//**************************************************************************
//
//   NST_UDT.AWL
//
//   PLC user interface assignment (810D/840D/840Di/FM-NC)
//
//   UDT  2 AL/MSG-UDT
//   UDT 10 NCK-UDT
//   UDT 11 BAG-UDT
//   UDT 19 MMC-UDT
//   UDT 21 Channel UDT
//   UDT 31 Axis/Spindle UDT
//   UDT 77 Mcp
//   UDT 1002 new Alarms
//
//**************************************************************************

//********** FM/BM-UDT **********
TYPE UDT 2


  STRUCT
   C1 : STRUCT  //From Channel 1
    FDD_5100xx : ARRAY  [0 .. 15 ] OF //Feed disable A.no.51000-510015
    BOOL ;
    FDD_RID_5101xx : ARRAY  [0 .. 31 ] OF //Feed and read-in disable A.no.510100-510131
    BOOL ;
    RID_5102xx : ARRAY  [0 .. 31 ] OF //Read-in disable A.no.510200-510231
    BOOL ;
    NCSD_5103xx : ARRAY  [0 .. 15 ] OF //NC start disable A.no.510300-510315
    BOOL ;
    FdStop_1_5111xx : ARRAY  [0 .. 15 ] OF //Feed stop GEOaxis 1 A.no.511100-511115
    BOOL ;
    FdStop_2_5112xx : ARRAY  [0 .. 15 ] OF //Feed stop GEOaxis 2 A.no.511200-511215
    BOOL ;
    FdStop_3_5113xx : ARRAY  [0 .. 15 ] OF //Feed stop GEOaxis 3 A.no.511300-511315
    BOOL ;
   END_STRUCT ;
   C2 : STRUCT  //From Channel 2
    FDD_5200xx : ARRAY  [0 .. 15 ] OF //Feed disable A.no.520000-520015
    BOOL ;
    FDD_RID_5201xx : ARRAY  [0 .. 31 ] OF //Feed and read-in disable A.no.520100-520131
    BOOL ;
    RID_5202xx : ARRAY  [0 .. 31 ] OF //Read-in disable A.no.520200-520231
    BOOL ;
    NCSD_5203xx : ARRAY  [0 .. 15 ] OF //NC start disable A.no.520300-520315
    BOOL ;
    FdStop_1_5211xx : ARRAY  [0 .. 15 ] OF //Feed stop GEOaxis 1 A.no.521100-521115
    BOOL ;
    FdStop_2_5212xx : ARRAY  [0 .. 15 ] OF //Feed stop GEOaxis 2 A.no.521200-521215
    BOOL ;
    FdStop_3_5213xx : ARRAY  [0 .. 15 ] OF //Feed stop GEOaxis 3 A.no.521300-521315
    BOOL ;
   END_STRUCT ;
   C3 : STRUCT  //From Channel 3
    FDD_5300xx : ARRAY  [0 .. 15 ] OF //Feed disable A.no.530000-530015
    BOOL ;
    FDD_RID_5301xx : ARRAY  [0 .. 31 ] OF //Feed and read-in disable A.no.530100-530131
    BOOL ;
    RID_5302xx : ARRAY  [0 .. 31 ] OF //Read-in disable A.no.530200-530231
    BOOL ;
    NCSD_5303xx : ARRAY  [0 .. 15 ] OF //NC start disable A.no.530300-530315
    BOOL ;
    FdStop_1_5311xx : ARRAY  [0 .. 15 ] OF //Feed stop GEOaxis 1 A.no.531100-531115
    BOOL ;
    FdStop_2_5312xx : ARRAY  [0 .. 15 ] OF //Feed stop GEOaxis 2 A.no.531200-531215
    BOOL ;
    FdStop_3_5313xx : ARRAY  [0 .. 15 ] OF //Feed stop GEOaxis 3 A.no.531300-531315
    BOOL ;
   END_STRUCT ;
   C4 : STRUCT  //From Channel 4
    FDD_5400xx : ARRAY  [0 .. 15 ] OF //Feed disable A.no.540000-540015
    BOOL ;
    FDD_RID_5401xx : ARRAY  [0 .. 31 ] OF //Feed and read-in disable A.no.540100-540131
    BOOL ;
    RID_5402xx : ARRAY  [0 .. 31 ] OF //Read-in disable A.no.540200-540231
    BOOL ;
    NCSD_5403xx : ARRAY  [0 .. 15 ] OF //NC start disable A.no.540300-540315
    BOOL ;
    FdStop_1_5411xx : ARRAY  [0 .. 15 ] OF //Feed stop GEOaxis 1 A.no.541100-541115
    BOOL ;
    FdStop_2_5412xx : ARRAY  [0 .. 15 ] OF //Feed stop GEOaxis 2 A.no.541200-541215
    BOOL ;
    FdStop_3_5413xx : ARRAY  [0 .. 15 ] OF //Feed stop GEOaxis 3 A.no.541300-541315
    BOOL ;
   END_STRUCT ;
   C5 : STRUCT  //From Channel 5
    FDD_5500xx : ARRAY  [0 .. 15 ] OF //Feed disable A.no.550000-550015
    BOOL ;
    FDD_RID_5501xx : ARRAY  [0 .. 31 ] OF //Feed and read-in disable A.no.550100-550131
    BOOL ;
    RID_5502xx : ARRAY  [0 .. 31 ] OF //Read-in disable A.no.550200-550231
    BOOL ;
    NCSD_5503xx : ARRAY  [0 .. 15 ] OF //NC start disable A.no.550300-550315
    BOOL ;
    FdStop_1_5511xx : ARRAY  [0 .. 15 ] OF //Feed stop GEOaxis 1 A.no.551100-551115
    BOOL ;
    FdStop_2_5512xx : ARRAY  [0 .. 15 ] OF //Feed stop GEOaxis 2 A.no.551200-551215
    BOOL ;
    FdStop_3_5513xx : ARRAY  [0 .. 15 ] OF //Feed stop GEOaxis 3 A.no.551300-551315
    BOOL ;
   END_STRUCT ;
   C6 : STRUCT  //From Channel 6
    FDD_5600xx : ARRAY  [0 .. 15 ] OF //Feed disable A.no.560000-560015
    BOOL ;
    FDD_RID_5601xx : ARRAY  [0 .. 31 ] OF //Feed and read-in disable A.no.560100-560131
    BOOL ;
    RID_5602xx : ARRAY  [0 .. 31 ] OF //Read-in disable A.no.560200-560231
    BOOL ;
    NCSD_5603xx : ARRAY  [0 .. 15 ] OF //NC start disable A.no.560300-560315
    BOOL ;
    FdStop_1_5611xx : ARRAY  [0 .. 15 ] OF //Feed stop GEOaxis 1 A.no.561100-561115
    BOOL ;
    FdStop_2_5612xx : ARRAY  [0 .. 15 ] OF //Feed stop GEOaxis 2 A.no.561200-561215
    BOOL ;
    FdStop_3_5613xx : ARRAY  [0 .. 15 ] OF //Feed stop GEOaxis 3 A.no.561300-561315
    BOOL ;
   END_STRUCT ;
   C7 : STRUCT  //From Channel 7
    FDD_5700xx : ARRAY  [0 .. 15 ] OF //Feed disable A.no.570000-570015
    BOOL ;
    FDD_RID_5701xx : ARRAY  [0 .. 31 ] OF //Feed and read-in disable A.no.570100-570131
    BOOL ;
    RID_5702xx : ARRAY  [0 .. 31 ] OF //Read-in disable A.no.570200-570231
    BOOL ;
    NCSD_5703xx : ARRAY  [0 .. 15 ] OF //NC start disable A.no.570300-570315
    BOOL ;
    FdStop_1_5711xx : ARRAY  [0 .. 15 ] OF //Feed stop GEOaxis 1 A.no.571100-511115
    BOOL ;
    FdStop_2_5712xx : ARRAY  [0 .. 15 ] OF //Feed stop GEOaxis 2 A.no.571200-511215
    BOOL ;
    FdStop_3_5713xx : ARRAY  [0 .. 15 ] OF //Feed stop GEOaxis 3 A.no.571300-511315
    BOOL ;
   END_STRUCT ;
   C8 : STRUCT  //From Channel 8
    FDD_5800xx : ARRAY  [0 .. 15 ] OF //Feed disable A.no.580000-580015
    BOOL ;
    FDD_RID_5801xx : ARRAY  [0 .. 31 ] OF //Feed and read-in disable A.no.580100-510131
    BOOL ;
    RID_5802xx : ARRAY  [0 .. 31 ] OF //Read-in disable A.no.580200-580231
    BOOL ;
    NCSD_5803xx : ARRAY  [0 .. 15 ] OF //NC start disable A.no.580300-580315
    BOOL ;
    FdStop_1_5811xx : ARRAY  [0 .. 15 ] OF //Feed stop GEOaxis 1 A.no.581100-511115
    BOOL ;
    FdStop_2_5812xx : ARRAY  [0 .. 15 ] OF //Feed stop GEOaxis 2 A.no.581200-511215
    BOOL ;
    FdStop_3_5813xx : ARRAY  [0 .. 15 ] OF //Feed stop GEOaxis 3 A.no.581300-511315
    BOOL ;
   END_STRUCT ;

    _1FdStop6001xx : ARRAY  [0 .. 15 ] OF //Feed stop axis/spindle 1
    BOOL ;
    _2FdStop6002xx : ARRAY  [0 .. 15 ] OF //Feed stop axis/spindle 2
    BOOL ;
    _3FdStop6003xx : ARRAY  [0 .. 15 ] OF //Feed stop axis/spindle 3
    BOOL ;
    _4FdStop6004xx : ARRAY  [0 .. 15 ] OF //Feed stop axis/spindle 4
    BOOL ;
    _5FdStop6005xx : ARRAY  [0 .. 15 ] OF //Feed stop axis/spindle 5
    BOOL ;
    _6FdStop6006xx : ARRAY  [0 .. 15 ] OF //Feed stop axis/spindle 6
    BOOL ;
    _7FdStop6007xx : ARRAY  [0 .. 15 ] OF //Feed stop axis/spindle 7
    BOOL ;
    _8FdStop6008xx : ARRAY  [0 .. 15 ] OF //Feed stop axis/spindle 8
    BOOL ;
    _9FdStop6009xx : ARRAY  [0 .. 15 ] OF //Feed stop axis/spindle 9
    BOOL ;
   _10FdStop6010xx : ARRAY  [0 .. 15 ] OF //Feed stop axis/spindle 10
    BOOL ;
   _11FdStop6011xx : ARRAY  [0 .. 15 ] OF //Feed stop axis/spindle 11
    BOOL ;
   _12FdStop6012xx : ARRAY  [0 .. 15 ] OF //Feed stop axis/spindle 12
    BOOL ;
   _13FdStop6013xx : ARRAY  [0 .. 15 ] OF //Feed stop axis/spindle 13
    BOOL ;
   _14FdStop6014xx : ARRAY  [0 .. 15 ] OF //Feed stop axis/spindle 14
    BOOL ;
   _15FdStop6015xx : ARRAY  [0 .. 15 ] OF //Feed stop axis/spindle 15
    BOOL ;
   _16FdStop6016xx : ARRAY  [0 .. 15 ] OF //Feed stop axis/spindle 16
    BOOL ;
   _17FdStop6017xx : ARRAY  [0 .. 15 ] OF //Feed stop axis/spindle 17
    BOOL ;
   _18FdStop6018xx : ARRAY  [0 .. 15 ] OF //Feed stop axis/spindle 18
    BOOL ;

   A7000xx : ARRAY  [0 .. 63 ] OF //Alarm 700000-700063 (user area 0)
   BOOL ;
   A7001xx : ARRAY  [0 .. 63 ] OF //Alarm 700100-700163 (user area 1)
   BOOL ;
   A7002xx : ARRAY  [0 .. 63 ] OF //Alarm 700200-700263 (user area 2)
   BOOL ;
   A7003xx : ARRAY  [0 .. 63 ] OF //Alarm 700300-700363 (user area 3)
   BOOL ;
   A7004xx : ARRAY  [0 .. 63 ] OF //Alarm 700400-700463 (user area 4)
   BOOL ;
   A7005xx : ARRAY  [0 .. 63 ] OF //Alarm 700500-700563 (user area 5
   BOOL ;
   A7006xx : ARRAY  [0 .. 63 ] OF //Alarm 700600-700663 (user area 6)
   BOOL ;
   A7007xx : ARRAY  [0 .. 63 ] OF //Alarm 700700-700763 (user area 7)
   BOOL ;
   A7008xx : ARRAY  [0 .. 63 ] OF //Alarm 700800-700863 (user area 8)
   BOOL ;
   A7009xx : ARRAY  [0 .. 63 ] OF //Alarm 700900-700963 (user area 9)
   BOOL ;
  END_STRUCT ;




END_TYPE


//********** NCK-UDT **********
TYPE UDT 10

    STRUCT
   A_Disabl_Inp1 : BOOL ;   //Disable digi. NCK input 1
   A_Disabl_Inp2 : BOOL ;   //Disable digi. NCK input 2
   A_Disabl_Inp3 : BOOL ;   //Disable digi. NCK input 3
   A_Disabl_Inp4 : BOOL ;   //Disable digi. NCK input 4
   A_Disabl_Inp5 : BOOL ;   //Disable digi. NCK input 5
   A_Disabl_Inp6 : BOOL ;   //Disable digi. NCK input 6
   A_Disabl_Inp7 : BOOL ;   //Disable digi. NCK input 7
   A_Disabl_Inp8 : BOOL ;   //Disable digi. NCK input 8
   A_Set_Inp1 : BOOL ;  //Set digi. NCK input 1
   A_Set_Inp2 : BOOL ;  //Set digi. NCK input 2
   A_Set_Inp3 : BOOL ;  //Set digi. NCK input 3
   A_Set_Inp4 : BOOL ;  //Set digi. NCK input 4
   A_Set_Inp5 : BOOL ;  //Set digi. NCK input 5
   A_Set_Inp6 : BOOL ;  //Set digi. NCK input 6
   A_Set_Inp7 : BOOL ;  //Set digi. NCK input 7
   A_Set_Inp8 : BOOL ;  //Set digi. NCK input 8
   f0_f15 : ARRAY  [0 .. 15 ] OF BOOL ; //Reserved
   A_Disabl_Out1 : BOOL ;   //Disable digi. NCK output 1
   A_Disabl_Out2 : BOOL ;   //Disable digi. NCK output 2
   A_Disabl_Out3 : BOOL ;   //Disable digi. NCK output 3
   A_Disabl_Out4 : BOOL ;   //Disable digi. NCK output 4
   A_Disabl_Out5 : BOOL ;   //Disable digi. NCK output 5
   A_Disabl_Out6 : BOOL ;   //Disable digi. NCK output 6
   A_Disabl_Out7 : BOOL ;   //Disable digi. NCK output 7
   A_Disabl_Out8 : BOOL ;   //Disable digi. NCK output 8
   A_OvMask_Out1 : BOOL ;   //Overwrite mask of digi. output 1
   A_OvMask_Out2 : BOOL ;   //Overwrite mask of digi. output 2
   A_OvMask_Out3 : BOOL ;   //Overwrite mask of digi. output 3
   A_OvMask_Out4 : BOOL ;   //Overwrite mask of digi. output 4
   A_OvMask_Out5 : BOOL ;   //Overwrite mask of digi. output 5
   A_OvMask_Out6 : BOOL ;   //Overwrite mask of digi. output 6
   A_OvMask_Out7 : BOOL ;   //Overwrite mask of digi. output 7
   A_OvMask_Out8 : BOOL ;   //Overwrite mask of digi. output 8
   A_Set_Out1 : BOOL ;  //Set digi. NCK output 1
   A_Set_Out2 : BOOL ;  //Set digi. NCK output 2
   A_Set_Out3 : BOOL ;  //Set digi. NCK output 3
   A_Set_Out4 : BOOL ;  //Set digi. NCK output 4
   A_Set_Out5 : BOOL ;  //Set digi. NCK output 5
   A_Set_Out6 : BOOL ;  //Set digi. NCK output 6
   A_Set_Out7 : BOOL ;  //Set digi. NCK output 7
   A_Set_Out8 : BOOL ;  //Set digi. NCK output 8
   A_InMask_Out1 : BOOL ;   //Input mask of digi. output 1
   A_InMask_Out2 : BOOL ;   //Input mask of digi. output 2
   A_InMask_Out3 : BOOL ;   //Input mask of digi. output 3
   A_InMask_Out4 : BOOL ;   //Input mask of digi. output 4
   A_InMask_Out5 : BOOL ;   //Input mask of digi. output 5
   A_InMask_Out6 : BOOL ;   //Input mask of digi. output 6
   A_InMask_Out7 : BOOL ;   //Input mask of digi. output 7
   A_InMask_Out8 : BOOL ;   //Input mask of digi. output 8
   MCP1AxisTbl : ARRAY  [1 .. 22 ] OF BYTE := B#16#1,B#16#2,B#16#3,B#16#4,B#16#5,B#16#6,B#16#7,
     B#16#8,B#16#9,B#16#0A,B#16#0B,B#16#0C ;    //Axis No. Table MCP1
   MCP1MaxAxis : Word ; //max. of Axisno, must be smaller or equal gp_par.MaxAxis
   MCP2AxisTbl : ARRAY  [1 .. 22 ] OF BYTE := B#16#1,B#16#2,B#16#3,B#16#4,B#16#5,B#16#6,B#16#7,
     B#16#8,B#16#9,B#16#0A,B#16#0B,B#16#0C ;    //Axis No. Table MCP2
   MCP2MaxAxis : Word ; //max. of Axisno, must be smaller or equal gp_par.MaxAxis
   f56_0 : BOOL ;
   A_EMERGENCY : BOOL ; //Emergency stop
   A_EMERGENCY_Ackn : BOOL ;    //Acknowledge emergency stop
   f56_3 : BOOL ;
   A_Keyswitch0 : BOOL ;    //Keyswitch position 0
   A_Keyswitch1 : BOOL ;    //Keyswitch position 1
   A_Keyswitch2 : BOOL ;    //Keyswitch position 2
   A_Keyswitch3 : BOOL ;    //Keyswitch position 3
   A_IncInModeGroup: BOOL ; //INC inputs in mode group area active
   f57_1 : BOOL ;
   f57_2 : BOOL ;
   A_PCshutdown : BOOL ;    //PC shutdown 840Di
   f57_4 : BOOL ;
   f57_5 : BOOL ;
   f57_6 : BOOL ;
   f57_7 : BOOL ;
   A_CollCheckOff: BOOL ; //Collisions Check Off
   f58_1 : BOOL ;
   f58_2 : BOOL ;
   f58_3 : BOOL ;
   f58_4 : BOOL ;
   f58_5 : BOOL ;
   f58_6 : BOOL ;
   f58_7 : BOOL ;
   f59 : BYTE ;
   E_ActVal_In1 : BOOL ;    //Actual value of digi. NCK input 1
   E_ActVal_In2 : BOOL ;    //Actual value of digi. NCK input 2
   E_ActVal_In3 : BOOL ;    //Actual value of digi. NCK input 3
   E_ActVal_In4 : BOOL ;    //Actual value of digi. NCK input 4
   f60_4 : BOOL ;
   f60_5 : BOOL ;
   f60_6 : BOOL ;
   f60_7 : BOOL ;
   f61_f62 : ARRAY  [61 .. 61 ] OF BYTE ;
   E_Setpoint_Out1 : BOOL ; //Setpoint of digi. NCK output 1
   E_Setpoint_Out2 : BOOL ; //Setpoint of digi. NCK output 2
   E_Setpoint_Out3 : BOOL ; //Setpoint of digi. NCK output 3
   E_Setpoint_Out4 : BOOL ; //Setpoint of digi. NCK output 4
   E_Setpoint_Out5 : BOOL ; //Setpoint of digi. NCK output 5
   E_Setpoint_Out6 : BOOL ; //Setpoint of digi. NCK output 6
   E_Setpoint_Out7 : BOOL ; //Setpoint of digi. NCK output 7
   E_Setpoint_Out8 : BOOL ; //Setpoint of digi. NCK output 8
   f65_f67 : ARRAY  [65 .. 66 ] OF BYTE ;
   E_HW1_moved : BYTE ; //Handwheel 1 moved
   E_HW2_moved : BYTE ; //Handwheel 2 moved
   E_HW3_moved : BYTE ; //Handwheel 3 moved
   E_CounterInchMetr : BYTE ;   //Modification counter inch/metric system of units

   E_MCP1AxisValid :Bool; //from HT6
   E_MCP1WCS :Bool; //from HT6
   f72_2: Bool;
   f72_3: Bool;
   f72_4: Bool;
   f72_5: Bool;
   f72_6: Bool;
   E_MCP1AxKeyDisp: Bool; //Mcp1 Axis Key Displayed
   E_MCP2AxisValid :Bool; //from HT6
   E_MCP2WCS :Bool; //from HT6
   f73_2: Bool;
   f73_3: Bool;
   f73_4: Bool;
   f73_5: Bool;
   f73_6: Bool;
   E_MCP2AxKeyDisp: Bool; //Mcp2 Axis Key Displayed
   MCP1AxisFromHMI : ARRAY [1..6] Of BYTE; //Axistable from HT6
   MCP2AxisFromHMI : ARRAY [1..6] Of BYTE; //Axistable from HT6
   res86 : Word;
   res88 : Byte;
   res89 : Byte;
   epsToPlc: Byte;
   epsFromPlc: Byte;
   MpiDpOk: BOOL;               //Slaves on MPI/DP Ok
   DpOk: BOOL;                  //Slaves on DP Ok
   PnOk : BOOL;                 //Slaves on PN Ok
   f92_3 : BOOL ;
   Disabl_AlarmMpiDp : BOOL;    //Disable Alarmmessage "MPI/DP bus error" (400551)
   Disabl_AlarmDp    : BOOL;    //Disable Alarmmessage "DP bus error" (400552)
   Disabl_AlarmPn    : BOOL;    //Disable Alarmmessage "PN bus error" (400553)
   f92_7 : BOOL ;
   E_CA_AutoMach  : BOOL;     // Disable collision avoidance : AUTO Machine
   E_CA_AutoTools : BOOL;     // Disable collision avoidance : AUTO Tools
   E_CA_AutoWorkh : BOOL;     // Disable collision avoidance : AUTO Workholder
   E_CA_AutoWorkp : BOOL;     // Disable collision avoidance : AUTO Workpieces
   E_CA_JogMach   : BOOL;     // Disable collision avoidance : JOG Machine
   E_CA_JogTools  : BOOL;     // Disable collision avoidance : JOG Tools
   E_CA_JogWorkh  : BOOL;     // Disable collision avoidance : JOG Workholder
   E_CA_JogWorkp  : BOOL;     // Disable collision avoidance : JOG Workpieces
   f94: BYTE ;
   f95: BYTE ;
   E_LanguageID : BYTE ;   // LanguageID on HMI
   E_Chan_HW1_A : BOOL ;    //Channel number for handwheel1 A
   E_Chan_HW1_B : BOOL ;    //Channel number for handwheel1 B
   E_Chan_HW1_C : BOOL ;    //Channel number for handwheel1 C
   E_Chan_HW1_D : BOOL ;    //Channel number for handwheel1 D
   f97_4 : BOOL ;
   f97_5 : BOOL ;
   f97_6 : BOOL ;
   f97_7 : BOOL ;
   E_Chan_HW2_A : BOOL ;    //Channel number for handwheel2 A
   E_Chan_HW2_B : BOOL ;    //Channel number for handwheel2 B
   E_Chan_HW2_C : BOOL ;    //Channel number for handwheel2 C
   E_Chan_HW2_D : BOOL ;    //Channel number for handwheel2 D
   f98_4 : BOOL ;
   f98_5 : BOOL ;
   f98_6 : BOOL ;
   f98_7 : BOOL ;
   E_Chan_HW3_A : BOOL ;    //Channel number for handwheel3 A
   E_Chan_HW3_B : BOOL ;    //Channel number for handwheel3 B
   E_Chan_HW3_C : BOOL ;    //Channel number for handwheel3 C
   E_Chan_HW3_D : BOOL ;    //Channel number for handwheel3 D
   f99_4 : BOOL ;
   f99_5 : BOOL ;
   f99_6 : BOOL ;
   f99_7 : BOOL ;
   E_Ax_A_HW1 : BOOL ;  //Axis number for handwheel1 A
   E_Ax_B_HW1 : BOOL ;  //Axis number for handwheel1 B
   E_Ax_C_HW1 : BOOL ;  //Axis number for handwheel1 C
   E_Ax_D_HW1 : BOOL ;  //Axis number for handwheel1 D
   E_Ax_E_HW1 : BOOL ;  //Axis number for handwheel1 E
   E_CHW_sel1 : BOOL ;  //Contour handwheel selected
   E_HW_sel1 : BOOL ;   //Handwheel selected
   E_Mach_Ax1 : BOOL ;  //Machine axis
   E_Ax_A_HW2 : BOOL ;  //Axis number for handwheel2 A
   E_Ax_B_HW2 : BOOL ;  //Axis number for handwheel2 B
   E_Ax_C_HW2 : BOOL ;  //Axis number for handwheel2 C
   E_Ax_D_HW2 : BOOL ;  //Axis number for handwheel2 D
   E_Ax_E_HW2 : BOOL ;  //Axis number for handwheel2 E
   E_CHW_sel2 : BOOL ;  //Contour handwheel selected
   E_HW_sel2 : BOOL ;   //Handwheel selected
   E_Mach_Ax2 : BOOL ;  //Machine axis
   E_Ax_A_HW3 : BOOL ;  //Axis number for handwheel3 A
   E_Ax_B_HW3 : BOOL ;  //Axis number for handwheel3 B
   E_Ax_C_HW3 : BOOL ;  //Axis number for handwheel3 C
   E_Ax_D_HW3 : BOOL ;  //Axis number for handwheel3 D
   E_Ax_E_HW3 : BOOL ;  //Axis number for handwheel3 E
   E_CHW_sel3 : BOOL ;  //Contour handwheel selected
   E_HW_sel3 : BOOL ;   //Handwheel selected
   E_Mach_Ax3 : BOOL ;  //Machine axis
   E_RemDiag : BOOL ;   //Remote Diagnostic
   f103_1 : BOOL ;
   f103_2 : BOOL ;
   f103_3 : BOOL ;
   f103_4 : BOOL ;
   E_ATready : BOOL ;   //AT-box ready
   E_MMCTemp : BOOL ;   //MMC temperature limit
   E_MMCBatt : BOOL ;   //MMC 101/102 battery alarm
   E_MCP1ready : BOOL ; //MCP1 ready;
   E_MCP2ready : BOOL ; //MCP2 ready;
   E_BHGready : BOOL ;  //BHG ready;
   f104_3 : BOOL ;
   f104_4 : BOOL ;
   f104_5 : BOOL ;
   E_FirstOB1 : BOOL ;  //This bit is on for the first OB1 cycle
   E_NCKready : BOOL ;  //NCK CPU ready
   E_CancelToolCmd : BOOL; //Terminate canceled tool command
   f105_1   : BOOL;
   f105_2   : BOOL;
   f105_3   : BOOL;
   f105_4   : BOOL;
   f105_5   : BOOL;
   f105_6   : BOOL;
   f105_7   : BOOL;
   E_CollCheckOff : BOOL ;  //CollisionsCheck Off
   E_EMSTOP : BOOL ;    //EMERGENCY STOP active
   f106_2 : BOOL ;
   f106_3 : BOOL ;
   f106_4 : BOOL ;
   f106_5 : BOOL ;
   f106_6 : BOOL ;
   f106_7 : BOOL ;
   E_InspProbe1 : BOOL ;    //Inspection probe 1 actuated
   E_InspProbe2 : BOOL ;    //Inspection probe 2 actuated
   f107_2 : BOOL ;
   f107_3 : BOOL ;
   f107_4 : BOOL ;
   f107_5 : BOOL ;
   E_NCU_LinkActive : BOOL ;    //NCU link active
   E_SystemInchDim : BOOL ; //System inch dimension
   f108_0 : BOOL ;
   E_MMC2Ready : BOOL ;     //MMC2-CPU ready
   E_MMCMPIready : BOOL ;   //MMC1-CPU on MPI ready
   E_MMCBTSSready : BOOL ;  //MMC1-CPU on BTSS ready
   f108_4 : BOOL ;
   E_DrivesInCylOp : BOOL ; //Drives in cylindric operation
   E_611Dready : BOOL ; //611D ready
   E_NCready : BOOL ;
   E_NCKalarm : BOOL ;  //NCK alarm present
   f109_1 : BOOL ;
   f109_2 : BOOL ;
   f109_3 : BOOL ;
   A_PC_OSfault : BOOL ;    //PC operating system fault, 840Di
   E_HTempAlarm : BOOL ;    //Heat sink temperature alarm NCU 573
   E_ATempAlarm : BOOL ;    //Air temperature alarm
   E_BattAlarm : BOOL ; //NCK battery alarm
   E_SWCamMinus : ARRAY  [0 .. 31 ] OF BOOL ;   //Software cams minus [0..31]
   E_SWCamPlus : ARRAY  [0 .. 31 ] OF BOOL ;    //Software cams plus [0..31]
   f118_f121 : ARRAY  [0 .. 3 ] OF BYTE ;
   A_Disabl_Inp9 : BOOL ;   //Disable digi. NCK input 9
   A_Disabl_Inp10 : BOOL ;  //Disable digi. NCK input 10
   A_Disabl_Inp11 : BOOL ;  //Disable digi. NCK input 11
   A_Disabl_Inp12 : BOOL ;  //Disable digi. NCK input 12
   A_Disabl_Inp13 : BOOL ;  //Disable digi. NCK input 13
   A_Disabl_Inp14 : BOOL ;  //Disable digi. NCK input 14
   A_Disabl_Inp15 : BOOL ;  //Disable digi. NCK input 15
   A_Disabl_Inp16 : BOOL ;  //Disable digi. NCK input 16
   A_Set_Inp9 : BOOL ;  //Set digi. NCK input 9
   A_Set_Inp10 : BOOL ; //Set digi. NCK input 10
   A_Set_Inp11 : BOOL ; //Set digi. NCK input 11
   A_Set_Inp12 : BOOL ; //Set digi. NCK input 12
   A_Set_Inp13 : BOOL ; //Set digi. NCK input 13
   A_Set_Inp14 : BOOL ; //Set digi. NCK input 14
   A_Set_Inp15 : BOOL ; //Set digi. NCK input 15
   A_Set_Inp16 : BOOL ; //Set digi. NCK input 16
   A_Disabl_Inp17 : BOOL ;  //Disable digi. NCK input 17
   A_Disabl_Inp18 : BOOL ;  //Disable digi. NCK input 18
   A_Disabl_Inp19 : BOOL ;  //Disable digi. NCK input 19
   A_Disabl_Inp20 : BOOL ;  //Disable digi. NCK input 20
   A_Disabl_Inp21 : BOOL ;  //Disable digi. NCK input 21
   A_Disabl_Inp22 : BOOL ;  //Disable digi. NCK input 22
   A_Disabl_Inp23 : BOOL ;  //Disable digi. NCK input 23
   A_Disabl_Inp24 : BOOL ;  //Disable digi. NCK input 24
   A_Set_Inp17 : BOOL ; //Set digi. NCK input 17
   A_Set_Inp18 : BOOL ; //Set digi. NCK input 18
   A_Set_Inp19 : BOOL ; //Set digi. NCK input 19
   A_Set_Inp20 : BOOL ; //Set digi. NCK input 20
   A_Set_Inp21 : BOOL ; //Set digi. NCK input 21
   A_Set_Inp22 : BOOL ; //Set digi. NCK input 22
   A_Set_Inp23 : BOOL ; //Set digi. NCK input 23
   A_Set_Inp24 : BOOL ; //Set digi. NCK input 24
   A_Disabl_Inp25 : BOOL ;  //Disable digi. NCK input 25
   A_Disabl_Inp26 : BOOL ;  //Disable digi. NCK input 26
   A_Disabl_Inp27 : BOOL ;  //Disable digi. NCK input 27
   A_Disabl_Inp28 : BOOL ;  //Disable digi. NCK input 28
   A_Disabl_Inp29 : BOOL ;  //Disable digi. NCK input 29
   A_Disabl_Inp30 : BOOL ;  //Disable digi. NCK input 30
   A_Disabl_Inp31 : BOOL ;  //Disable digi. NCK input 31
   A_Disabl_Inp32 : BOOL ;  //Disable digi. NCK input 32
   A_Set_Inp25 : BOOL ; //Set digi. NCK input 25
   A_Set_Inp26 : BOOL ; //Set digi. NCK input 26
   A_Set_Inp27 : BOOL ; //Set digi. NCK input 27
   A_Set_Inp28 : BOOL ; //Set digi. NCK input 28
   A_Set_Inp29 : BOOL ; //Set digi. NCK input 29
   A_Set_Inp30 : BOOL ; //Set digi. NCK input 30
   A_Set_Inp31 : BOOL ; //Set digi. NCK input 31
   A_Set_Inp32 : BOOL ; //Set digi. NCK input 32
   A_Disabl_Inp33 : BOOL ;  //Disable digi. NCK input 33
   A_Disabl_Inp34 : BOOL ;  //Disable digi. NCK input 34
   A_Disabl_Inp35 : BOOL ;  //Disable digi. NCK input 35
   A_Disabl_Inp36 : BOOL ;  //Disable digi. NCK input 36
   A_Disabl_Inp37 : BOOL ;  //Disable digi. NCK input 37
   A_Disabl_Inp38 : BOOL ;  //Disable digi. NCK input 38
   A_Disabl_Inp39 : BOOL ;  //Disable digi. NCK input 39
   A_Disabl_Inp40 : BOOL ;  //Disable digi. NCK input 40
   A_Set_Inp33 : BOOL ; //Set digi. NCK input 33
   A_Set_Inp34 : BOOL ; //Set digi. NCK input 34
   A_Set_Inp35 : BOOL ; //Set digi. NCK input 35
   A_Set_Inp36 : BOOL ; //Set digi. NCK input 36
   A_Set_Inp37 : BOOL ; //Set digi. NCK input 37
   A_Set_Inp38 : BOOL ; //Set digi. NCK input 38
   A_Set_Inp39 : BOOL ; //Set digi. NCK input 39
   A_Set_Inp40 : BOOL ; //Set digi. NCK input 40
   A_Disabl_Out9 : BOOL ;   //Disable digi. NCK output 9
   A_Disabl_Out10 : BOOL ;  //Disable digi. NCK output 10
   A_Disabl_Out11 : BOOL ;  //Disable digi. NCK output 11
   A_Disabl_Out12 : BOOL ;  //Disable digi. NCK output 12
   A_Disabl_Out13 : BOOL ;  //Disable digi. NCK output 13
   A_Disabl_Out14 : BOOL ;  //Disable digi. NCK output 14
   A_Disabl_Out15 : BOOL ;  //Disable digi. NCK output 15
   A_Disabl_Out16 : BOOL ;  //Disable digi. NCK output 16
   A_OvMask_Out9 : BOOL ;   //Overwrite mask of digi. output 9
   A_OvMask_Out10 : BOOL ;  //Overwrite mask of digi. output 10
   A_OvMask_Out11 : BOOL ;  //Overwrite mask of digi. output 11
   A_OvMask_Out12 : BOOL ;  //Overwrite mask of digi. output 12
   A_OvMask_Out13 : BOOL ;  //Overwrite mask of digi. output 13
   A_OvMask_Out14 : BOOL ;  //Overwrite mask of digi. output 14
   A_OvMask_Out15 : BOOL ;  //Overwrite mask of digi. output 15
   A_OvMask_Out16 : BOOL ;  //Overwrite mask of digi. output 16
   A_Setval_Out9 : BOOL ;   //Set value digi. NCK output 9
   A_Setval_Out10 : BOOL ;  //Set value digi. NCK output 10
   A_Setval_Out11 : BOOL ;  //Set value digi. NCK output 11
   A_Setval_Out12 : BOOL ;  //Set value digi. NCK output 12
   A_Setval_Out13 : BOOL ;  //Set value digi. NCK output 13
   A_Setval_Out14 : BOOL ;  //Set value digi. NCK output 14
   A_Setval_Out15 : BOOL ;  //Set value digi. NCK output 15
   A_Setval_Out16 : BOOL ;  //Set value digi. NCK output 16
   A_InMask_Out9 : BOOL ;   //Input mask of digi. output 9
   A_InMask_Out10 : BOOL ;  //Input mask of digi. output 10
   A_InMask_Out11 : BOOL ;  //Input mask of digi. output 11
   A_InMask_Out12 : BOOL ;  //Input mask of digi. output 12
   A_InMask_Out13 : BOOL ;  //Input mask of digi. output 13
   A_InMask_Out14 : BOOL ;  //Input mask of digi. output 14
   A_InMask_Out15 : BOOL ;  //Input mask of digi. output 15
   A_InMask_Out16 : BOOL ;  //Input mask of digi. output 16
   A_Disabl_Out17 : BOOL ;  //Disable digi. NCK output 17
   A_Disabl_Out18 : BOOL ;  //Disable digi. NCK output 18
   A_Disabl_Out19 : BOOL ;  //Disable digi. NCK output 19
   A_Disabl_Out20 : BOOL ;  //Disable digi. NCK output 20
   A_Disabl_Out21 : BOOL ;  //Disable digi. NCK output 21
   A_Disabl_Out22 : BOOL ;  //Disable digi. NCK output 22
   A_Disabl_Out23 : BOOL ;  //Disable digi. NCK output 23
   A_Disabl_Out24 : BOOL ;  //Disable digi. NCK output 24
   A_OvMask_Out17 : BOOL ;  //Overwrite mask of digi. output 17
   A_OvMask_Out18 : BOOL ;  //Overwrite mask of digi. output 18
   A_OvMask_Out19 : BOOL ;  //Overwrite mask of digi. output 19
   A_OvMask_Out20 : BOOL ;  //Overwrite mask of digi. output 20
   A_OvMask_Out21 : BOOL ;  //Overwrite mask of digi. output 21
   A_OvMask_Out22 : BOOL ;  //Overwrite mask of digi. output 22
   A_OvMask_Out23 : BOOL ;  //Overwrite mask of digi. output 23
   A_OvMask_Out24 : BOOL ;  //Overwrite mask of digi. output 24
   A_Setval_Out17 : BOOL ;  //Set value digi. NCK output 17
   A_Setval_Out18 : BOOL ;  //Set value digi. NCK output 18
   A_Setval_Out19 : BOOL ;  //Set value digi. NCK output 19
   A_Setval_Out20 : BOOL ;  //Set value digi. NCK output 20
   A_Setval_Out21 : BOOL ;  //Set value digi. NCK output 21
   A_Setval_Out22 : BOOL ;  //Set value digi. NCK output 22
   A_Setval_Out23 : BOOL ;  //Set value digi. NCK output 23
   A_Setval_Out24 : BOOL ;  //Set value digi. NCK output 24
   A_InMask_Out17 : BOOL ;  //Input mask of digi. output 17
   A_InMask_Out18 : BOOL ;  //Input mask of digi. output 18
   A_InMask_Out19 : BOOL ;  //Input mask of digi. output 19
   A_InMask_Out20 : BOOL ;  //Input mask of digi. output 20
   A_InMask_Out21 : BOOL ;  //Input mask of digi. output 21
   A_InMask_Out22 : BOOL ;  //Input mask of digi. output 22
   A_InMask_Out23 : BOOL ;  //Input mask of digi. output 23
   A_InMask_Out24 : BOOL ;  //Input mask of digi. output 24
   A_Disabl_Out25 : BOOL ;  //Disable digi. NCK output 25
   A_Disabl_Out26 : BOOL ;  //Disable digi. NCK output 26
   A_Disabl_Out27 : BOOL ;  //Disable digi. NCK output 27
   A_Disabl_Out28 : BOOL ;  //Disable digi. NCK output 28
   A_Disabl_Out29 : BOOL ;  //Disable digi. NCK output 29
   A_Disabl_Out30 : BOOL ;  //Disable digi. NCK output 30
   A_Disabl_Out31 : BOOL ;  //Disable digi. NCK output 31
   A_Disabl_Out32 : BOOL ;  //Disable digi. NCK output 32
   A_OvMask_Out25 : BOOL ;  //Overwrite mask of digi. output 25
   A_OvMask_Out26 : BOOL ;  //Overwrite mask of digi. output 26
   A_OvMask_Out27 : BOOL ;  //Overwrite mask of digi. output 27
   A_OvMask_Out28 : BOOL ;  //Overwrite mask of digi. output 28
   A_OvMask_Out29 : BOOL ;  //Overwrite mask of digi. output 29
   A_OvMask_Out30 : BOOL ;  //Overwrite mask of digi. output 30
   A_OvMask_Out31 : BOOL ;  //Overwrite mask of digi. output 31
   A_OvMask_Out32 : BOOL ;  //Overwrite mask of digi. output 32
   A_Setval_Out25 : BOOL ;  //Set value digi. NCK output 25
   A_Setval_Out26 : BOOL ;  //Set value digi. NCK output 26
   A_Setval_Out27 : BOOL ;  //Set value digi. NCK output 27
   A_Setval_Out28 : BOOL ;  //Set value digi. NCK output 28
   A_Setval_Out29 : BOOL ;  //Set value digi. NCK output 29
   A_Setval_Out30 : BOOL ;  //Set value digi. NCK output 30
   A_Setval_Out31 : BOOL ;  //Set value digi. NCK output 31
   A_Setval_Out32 : BOOL ;  //Set value digi. NCK output 32
   A_InMask_Out25 : BOOL ;  //Input mask of digi. output 25
   A_InMask_Out26 : BOOL ;  //Input mask of digi. output 26
   A_InMask_Out27 : BOOL ;  //Input mask of digi. output 27
   A_InMask_Out28 : BOOL ;  //Input mask of digi. output 28
   A_InMask_Out29 : BOOL ;  //Input mask of digi. output 29
   A_InMask_Out30 : BOOL ;  //Input mask of digi. output 30
   A_InMask_Out31 : BOOL ;  //Input mask of digi. output 31
   A_InMask_Out32 : BOOL ;  //Input mask of digi. output 32
   A_Disabl_Out33 : BOOL ;  //Disable digi. NCK output 33
   A_Disabl_Out34 : BOOL ;  //Disable digi. NCK output 34
   A_Disabl_Out35 : BOOL ;  //Disable digi. NCK output 35
   A_Disabl_Out36 : BOOL ;  //Disable digi. NCK output 36
   A_Disabl_Out37 : BOOL ;  //Disable digi. NCK output 37
   A_Disabl_Out38 : BOOL ;  //Disable digi. NCK output 38
   A_Disabl_Out39 : BOOL ;  //Disable digi. NCK output 39
   A_Disabl_Out40 : BOOL ;  //Disable digi. NCK output 40
   A_OvMask_Out33 : BOOL ;  //Overwrite mask of digi. output 33
   A_OvMask_Out34 : BOOL ;  //Overwrite mask of digi. output 34
   A_OvMask_Out35 : BOOL ;  //Overwrite mask of digi. output 35
   A_OvMask_Out36 : BOOL ;  //Overwrite mask of digi. output 36
   A_OvMask_Out37 : BOOL ;  //Overwrite mask of digi. output 37
   A_OvMask_Out38 : BOOL ;  //Overwrite mask of digi. output 38
   A_OvMask_Out39 : BOOL ;  //Overwrite mask of digi. output 39
   A_OvMask_Out40 : BOOL ;  //Overwrite mask of digi. output 40
   A_Setval_out33 : BOOL ;  //Set value digi. NCK output 33
   A_Setval_out34 : BOOL ;  //Set value digi. NCK output 34
   A_Setval_out35 : BOOL ;  //Set value digi. NCK output 35
   A_Setval_out36 : BOOL ;  //Set value digi. NCK output 36
   A_Setval_out37 : BOOL ;  //Set value digi. NCK output 37
   A_Setval_out38 : BOOL ;  //Set value digi. NCK output 38
   A_Setval_out39 : BOOL ;  //Set value digi. NCK output 39
   A_Setval_out40 : BOOL ;  //Set value digi. NCK output 40
   A_InMask_Out33 : BOOL ;  //Input mask of digi. output 33
   A_InMask_Out34 : BOOL ;  //Input mask of digi. output 34
   A_InMask_Out35 : BOOL ;  //Input mask of digi. output 35
   A_InMask_Out36 : BOOL ;  //Input mask of digi. output 36
   A_InMask_Out37 : BOOL ;  //Input mask of digi. output 37
   A_InMask_Out38 : BOOL ;  //Input mask of digi. output 38
   A_InMask_Out39 : BOOL ;  //Input mask of digi. output 39
   A_InMask_Out40 : BOOL ;  //Input mask of digi. output 40
   A_Disabl_anaIn1 : BOOL ; //Disable analog NCK input 1
   A_Disabl_anaIn2 : BOOL ; //Disable analog NCK input 2
   A_Disabl_anaIn3 : BOOL ; //Disable analog NCK input 3
   A_Disabl_anaIn4 : BOOL ; //Disable analog NCK input 4
   A_Disabl_anaIn5 : BOOL ; //Disable analog NCK input 5
   A_Disabl_anaIn6 : BOOL ; //Disable analog NCK input 6
   A_Disabl_anaIn7 : BOOL ; //Disable analog NCK input 7
   A_Disabl_anaIn8 : BOOL ; //Disable analog NCK input 8
   A_InMask_anaIn1 : BOOL ; //Input mask of analog NCK input 1
   A_InMask_anaIn2 : BOOL ; //Input mask of analog NCK input 2
   A_InMask_anaIn3 : BOOL ; //Input mask of analog NCK input 3
   A_InMask_anaIn4 : BOOL ; //Input mask of analog NCK input 4
   A_InMask_anaIn5 : BOOL ; //Input mask of analog NCK input 5
   A_InMask_anaIn6 : BOOL ; //Input mask of analog NCK input 6
   A_InMask_anaIn7 : BOOL ; //Input mask of analog NCK input 7
   A_InMask_anaIn8 : BOOL ; //Input mask of analog NCK input 8
   A_Setval_anaIn1 : WORD ; //Set value of analog NCK input 1
   A_Setval_anaIn2 : WORD ; //Set value of analog NCK input 2
   A_Setval_anaIn3 : WORD ; //Set value of analog NCK input 3
   A_Setval_anaIn4 : WORD ; //Set value of analog NCK input 4
   A_Setval_anaIn5 : WORD ; //Set value of analog NCK input 5
   A_Setval_anaIn6 : WORD ; //Set value of analog NCK input 6
   A_Setval_anaIn7 : WORD ; //Set value of analog NCK input 7
   A_Setval_anaIn8 : WORD ; //Set value of analog NCK input 8
   f164_f165 : INT ;
   A_OvMask_anaOut1 : BOOL ;    //Overwrite mask of analog output 1
   A_OvMask_anaOut2 : BOOL ;    //Overwrite mask of analog output 2
   A_OvMask_anaOut3 : BOOL ;    //Overwrite mask of analog output 3
   A_OvMask_anaOut4 : BOOL ;    //Overwrite mask of analog output 4
   A_OvMask_anaOut5 : BOOL ;    //Overwrite mask of analog output 5
   A_OvMask_anaOut6 : BOOL ;    //Overwrite mask of analog output 6
   A_OvMask_anaOut7 : BOOL ;    //Overwrite mask of analog output 7
   A_OvMask_anaOut8 : BOOL ;    //Overwrite mask of analog output 8
   A_InMask_anaOut1 : BOOL ;    //Input mask of analog NCK output 1
   A_InMask_anaOut2 : BOOL ;    //Input mask of analog NCK output 2
   A_InMask_anaOut3 : BOOL ;    //Input mask of analog NCK output 3
   A_InMask_anaOut4 : BOOL ;    //Input mask of analog NCK output 4
   A_InMask_anaOut5 : BOOL ;    //Input mask of analog NCK output 5
   A_InMask_anaOut6 : BOOL ;    //Input mask of analog NCK output 6
   A_InMask_anaOut7 : BOOL ;    //Input mask of analog NCK output 7
   A_InMask_anaOut8 : BOOL ;    //Input mask of analog NCK output 8
   A_Disabl_anaOut1 : BOOL ;    //Disable analog NCK output 1
   A_Disabl_anaOut2 : BOOL ;    //Disable analog NCK output 2
   A_Disabl_anaOut3 : BOOL ;    //Disable analog NCK output 3
   A_Disabl_anaOut4 : BOOL ;    //Disable analog NCK output 4
   A_Disabl_anaOut5 : BOOL ;    //Disable analog NCK output 5
   A_Disabl_anaOut6 : BOOL ;    //Disable analog NCK output 6
   A_Disabl_anaOut7 : BOOL ;    //Disable analog NCK output 7
   A_Disabl_anaOut8 : BOOL ;    //Disable analog NCK output 8
   f169 : BYTE ;
   A_Setval_anaOut1 : WORD ;    //Set value of analog NCK output 1
   A_Setval_anaOut2 : WORD ;    //Set value of analog NCK output 2
   A_Setval_anaOut3 : WORD ;    //Set value of analog NCK output 3
   A_Setval_anaOut4 : WORD ;    //Set value of analog NCK output 4
   A_Setval_anaOut5 : WORD ;    //Set value of analog NCK output 5
   A_Setval_anaOut6 : WORD ;    //Set value of analog NCK output 6
   A_Setval_anaOut7 : WORD ;    //Set value of analog NCK output 7
   A_Setval_anaOut8 : WORD ;    //Set value of analog NCK output 8
   E_ActVal_In9 : BOOL ;    //Actual value of digi. NCK input 9
   E_ActVal_In10 : BOOL ;   //Actual value of digi. NCK input 10
   E_ActVal_In11 : BOOL ;   //Actual value of digi. NCK input 11
   E_ActVal_In12 : BOOL ;   //Actual value of digi. NCK input 12
   E_ActVal_In13 : BOOL ;   //Actual value of digi. NCK input 13
   E_ActVal_In14 : BOOL ;   //Actual value of digi. NCK input 14
   E_ActVal_In15 : BOOL ;   //Actual value of digi. NCK input 15
   E_ActVal_In16 : BOOL ;   //Actual value of digi. NCK input 16
   E_ActVal_In17 : BOOL ;   //Actual value of digi. NCK input 17
   E_ActVal_In18 : BOOL ;   //Actual value of digi. NCK input 18
   E_ActVal_In19 : BOOL ;   //Actual value of digi. NCK input 19
   E_ActVal_In20 : BOOL ;   //Actual value of digi. NCK input 20
   E_ActVal_In21 : BOOL ;   //Actual value of digi. NCK input 21
   E_ActVal_In22 : BOOL ;   //Actual value of digi. NCK input 22
   E_ActVal_In23 : BOOL ;   //Actual value of digi. NCK input 23
   E_ActVal_In24 : BOOL ;   //Actual value of digi. NCK input 24
   E_ActVal_In25 : BOOL ;   //Actual value of digi. NCK input 25
   E_ActVal_In26 : BOOL ;   //Actual value of digi. NCK input 26
   E_ActVal_In27 : BOOL ;   //Actual value of digi. NCK input 27
   E_ActVal_In28 : BOOL ;   //Actual value of digi. NCK input 28
   E_ActVal_In29 : BOOL ;   //Actual value of digi. NCK input 29
   E_ActVal_In30 : BOOL ;   //Actual value of digi. NCK input 30
   E_ActVal_In31 : BOOL ;   //Actual value of digi. NCK input 31
   E_ActVal_In32 : BOOL ;   //Actual value of digi. NCK input 32
   E_ActVal_In33 : BOOL ;   //Actual value of digi. NCK input 33
   E_ActVal_In34 : BOOL ;   //Actual value of digi. NCK input 34
   E_ActVal_In35 : BOOL ;   //Actual value of digi. NCK input 35
   E_ActVal_In36 : BOOL ;   //Actual value of digi. NCK input 36
   E_ActVal_In37 : BOOL ;   //Actual value of digi. NCK input 37
   E_ActVal_In38 : BOOL ;   //Actual value of digi. NCK input 38
   E_ActVal_In39 : BOOL ;   //Actual value of digi. NCK input 39
   E_ActVal_In40 : BOOL ;   //Actual value of digi. NCK input 40
   E_Setpoint_Out9 : BOOL ; //Setpoint of digi. NCK output 9
   E_Setpoint_Out10 : BOOL ;    //Setpoint of digi. NCK output 10
   E_Setpoint_Out11 : BOOL ;    //Setpoint of digi. NCK output 11
   E_Setpoint_Out12 : BOOL ;    //Setpoint of digi. NCK output 12
   E_Setpoint_Out13 : BOOL ;    //Setpoint of digi. NCK output 13
   E_Setpoint_Out14 : BOOL ;    //Setpoint of digi. NCK output 14
   E_Setpoint_Out15 : BOOL ;    //Setpoint of digi. NCK output 15
   E_Setpoint_Out16 : BOOL ;    //Setpoint of digi. NCK output 16
   E_Setpoint_Out17 : BOOL ;    //Setpoint of digi. NCK output 17
   E_Setpoint_Out18 : BOOL ;    //Setpoint of digi. NCK output 18
   E_Setpoint_Out19 : BOOL ;    //Setpoint of digi. NCK output 19
   E_Setpoint_Out20 : BOOL ;    //Setpoint of digi. NCK output 20
   E_Setpoint_Out21 : BOOL ;    //Setpoint of digi. NCK output 21
   E_Setpoint_Out22 : BOOL ;    //Setpoint of digi. NCK output 22
   E_Setpoint_Out23 : BOOL ;    //Setpoint of digi. NCK output 23
   E_Setpoint_Out24 : BOOL ;    //Setpoint of digi. NCK output 24
   E_Setpoint_Out25 : BOOL ;    //Setpoint of digi. NCK output 25
   E_Setpoint_Out26 : BOOL ;    //Setpoint of digi. NCK output 26
   E_Setpoint_Out27 : BOOL ;    //Setpoint of digi. NCK output 27
   E_Setpoint_Out28 : BOOL ;    //Setpoint of digi. NCK output 28
   E_Setpoint_Out29 : BOOL ;    //Setpoint of digi. NCK output 29
   E_Setpoint_Out30 : BOOL ;    //Setpoint of digi. NCK output 30
   E_Setpoint_Out31 : BOOL ;    //Setpoint of digi. NCK output 31
   E_Setpoint_Out32 : BOOL ;    //Setpoint of digi. NCK output 32
   E_Setpoint_Out33 : BOOL ;    //Setpoint of digi. NCK output 33
   E_Setpoint_Out34 : BOOL ;    //Setpoint of digi. NCK output 34
   E_Setpoint_Out35 : BOOL ;    //Setpoint of digi. NCK output 35
   E_Setpoint_Out36 : BOOL ;    //Setpoint of digi. NCK output 36
   E_Setpoint_Out37 : BOOL ;    //Setpoint of digi. NCK output 37
   E_Setpoint_Out38 : BOOL ;    //Setpoint of digi. NCK output 38
   E_Setpoint_Out39 : BOOL ;    //Setpoint of digi. NCK output 39
   E_Setpoint_Out40 : BOOL ;    //Setpoint of digi. NCK output 40
   E_ActVal_anaIn1 : WORD ; //Actual value of analog NCK input 1
   E_ActVal_anaIn2 : WORD ; //Actual value of analog NCK input 2
   E_ActVal_anaIn3 : WORD ; //Actual value of analog NCK input 3
   E_ActVal_anaIn4 : WORD ; //Actual value of analog NCK input 4
   E_ActVal_anaIn5 : WORD ; //Actual value of analog NCK input 5
   E_ActVal_anaIn6 : WORD ; //Actual value of analog NCK input 6
   E_ActVal_anaIn7 : WORD ; //Actual value of analog NCK input 7
   E_ActVal_anaIn8 : WORD ; //Actual value of analog NCK input 8
   E_SetVal_anaOut1 : WORD ;    //Set value of analog NCK output 1
   E_SetVal_anaOut2 : WORD ;    //Set value of analog NCK output 2
   E_SetVal_anaOut3 : WORD ;    //Set value of analog NCK output 3
   E_SetVal_anaOut4 : WORD ;    //Set value of analog NCK output 4
   E_SetVal_anaOut5 : WORD ;    //Set value of analog NCK output 5
   E_SetVal_anaOut6 : WORD ;    //Set value of analog NCK output 6
   E_SetVal_anaOut7 : WORD ;    //Set value of analog NCK output 7
   E_SetVal_anaOut8 : WORD ;    //Set value of analog NCK output 8
   E_CollCheck: ARRAY  [0 .. 7 ] OF BYTE ; //CollisionsCheck
   A_CollCheck: ARRAY  [0 .. 7 ] OF BYTE ; //CollisionsCheck

   E_HW4_moved    : BYTE ; //Handwheel 4 moved
   E_HW5_moved    : BYTE ; //Handwheel 5 moved
   E_HW6_moved    : BYTE ; //Handwheel 6 moved
   E_EHW1_stands  : BOOL;  //Ethernet handwheel 1 stands
   E_EHW2_stands  : BOOL;  //Ethernet handwheel 2 stands
   E_EHW3_stands  : BOOL;  //Ethernet handwheel 3 stands
   E_EHW4_stands  : BOOL;  //Ethernet handwheel 4 stands
   E_EHW5_stands  : BOOL;  //Ethernet handwheel 5 stands
   E_EHW6_stands  : BOOL;  //Ethernet handwheel 6 stands
   f245_6         : BOOL;
   f245_7         : BOOL;
   f246           : WORD;

   A_RobotStatus    : ARRAY [0 .. 7] OF BYTE;   //Robot Status
   E_RobotControl   : ARRAY [0 .. 7] OF BYTE;   //Robot Control
  END_STRUCT ;


END_TYPE


//********** BAG-UDT **********
TYPE UDT 11

    STRUCT
   A_AUTO : BOOL ;  //AUTOMATIC mode
   A_MDA : BOOL ;   //MDA mode
   A_JOG : BOOL ;   //JOG mode
   f0_3 : BOOL ;
   A_MCDisable : BOOL ; //Mode change disable
   A_MGStop : BOOL ;    //Mode group stop
   A_MGStopASp : BOOL ; //Mode group stop axes plus spindle
   A_MGReset : BOOL ;   //Mode group reset
   A_TEACHIN : BOOL ;   //Machine function TEACH IN
   A_REPOS : BOOL ; //Machine function REPOS
   A_REF : BOOL ;   //Machine function REF
   f1_3 : BOOL ;
   f1_4 : BOOL ;
   f1_5 : BOOL ;
   A_SingleBlock_B : BOOL ; // Single block type B
   A_SingleBlock_A : BOOL ; // Single block type A
   A_INC1 : BOOL ;  //INC1
   A_INC10 : BOOL ; //INC10
   A_INC100 : BOOL ;    //INC100
   A_INC1000 : BOOL ;   //INC1000
   A_INC10000 : BOOL ;  //INC10000
   A_INCVar : BOOL ;    //INC variable
   f3 : BYTE ;
   E_MMC_AUTO : BOOL ;  //MMC Strobe AUTOMATIC mode
   E_MMC_MDA : BOOL ;   //MMC Strobe MDA mode
   E_MMC_JOG : BOOL ;   //MMC Strobe JOG mode
   f4_3 : BOOL ;
   f4_4 : BOOL ;
   f4_5 : BOOL ;
   f4_6 : BOOL ;
   f4_7 : BOOL ;
   E_MMC_TEACHIN : BOOL ;   //MMC Strobe machine function TEACH IN
   E_MMC_REPOS : BOOL ; //MMC Strobe machine function REPOS
   E_MMC_REF : BOOL ;   //MMC Strobe Machine function REF
   f5_3 : BOOL ;
   f5_4 : BOOL ;
   f5_5 : BOOL ;
   f5_6 : BOOL ;
   f5_7 : BOOL ;
   E_AUTO : BOOL ;  //Active AUTOMATIC mode
   E_MDA : BOOL ;   //Active MDA mode
   E_JOG : BOOL ;   //Active JOG mode
   E_MGOK : BOOL ;  //Mode group ready
   E_MGreseted : BOOL ; // Mode Group reseted
   E_NCKintJOG : BOOL ; // NCK internal JOG active
   f6_6 : BOOL ;
   E_ChanReset : BOOL ; //All channels in reset state
   E_TEACHIN : BOOL ;   //Active machine function TEACH IN
   E_REPOS : BOOL ; //Active machine function REPOS
   E_REF : BOOL ;   //Active Machine function REF
   f7_3 : BOOL;
   f7_4 : BOOL;
   f7_5 : BOOL;
   f7_6 : BOOL;
   f7_7 : BOOL;
   E_INC1 : BOOL ;      // INC1
   E_INC10 : BOOL ;     // INC10
   E_INC100 : BOOL ;    // INC100
   E_INC1000 : BOOL ;   // INC1000
   E_INC10000 : BOOL ;  // INC10000
   E_INCVar : BOOL ;    // INC variable
   f8_6 : BOOL;
   f8_7 : BOOL;
   f9 : BYTE ;
   f10 : ARRAY  [10 .. 19 ] OF BYTE ;
   MG : ARRAY  [2 .. 10 ] OF STRUCT
    A_AUTO : BOOL ; //AUTOMATIC mode
    A_MDA : BOOL ;  //MDA mode
    A_JOG : BOOL ;  //JOG mode
    f0_3 : BOOL ;
    A_MCDisable : BOOL ;    //Mode change disable
    A_MGStop : BOOL ;   //Mode group stop
    A_MGStopASp : BOOL ;    //Mode group stop axes plus spindle
    A_MGReset : BOOL ;  //Mode group reset
    A_TEACHIN : BOOL ;  //Machine function TEACH IN
    A_REPOS : BOOL ;    //Machine function REPOS
    A_REF : BOOL ;  //Machine function REF
    f1_3 : BOOL ;
    f1_4 : BOOL ;
    f1_5 : BOOL ;
    A_SingleBlock_B : BOOL ; // Single block type B
    A_SingleBlock_A : BOOL ; // Single block type A
    A_INC1 : BOOL ; //INC1
    A_INC10 : BOOL ;    //INC10
    A_INC100 : BOOL ;   //INC100
    A_INC1000 : BOOL ;  //INC1000
    A_INC10000 : BOOL ; //INC10000
    A_INCVar : BOOL ;   //INC variable
    f3 : BYTE ;
    E_MMC_AUTO : BOOL ; //MMC Strobe AUTOMATIC mode
    E_MMC_MDA : BOOL ;  //MMC Strobe MDA mode
    E_MMC_JOG : BOOL ;  //MMC Strobe JOG mode
    f4_3 : BOOL ;
    f4_4 : BOOL ;
    f4_5 : BOOL ;
    f4_6 : BOOL ;
    f4_7 : BOOL ;
    E_MMC_TEACHIN : BOOL ;  //MMC Strobe machine function TEACH IN
    E_MMC_REPOS : BOOL ;    //MMC Strobe machine function REPOS
    E_MMC_REF : BOOL ;  //MMC Strobe Machine function REF
    f5_3 : BOOL ;
    f5_4 : BOOL ;
    f5_5 : BOOL ;
    f5_6 : BOOL ;
    f5_7 : BOOL ;
    E_AUTO : BOOL ; //Active AUTOMATIC mode
    E_MDA : BOOL ;  //Active MDA mode
    E_JOG : BOOL ;  //Active JOG mode
    E_MGOK : BOOL ; //Mode group ready
    E_MGreseted : BOOL ; // Mode Group reseted
    E_NCKintJOG : BOOL ; // NCK internal JOG active
    f6_6 : BOOL ;
    E_ChanReset : BOOL ;    //All channels in reset state
    E_TEACHIN : BOOL ;  //Active machine function TEACH IN
    E_REPOS : BOOL ;    //Active machine function REPOS
    E_REF : BOOL ;  //Active machine function REF
    f7_3 : BOOL;
    f7_4 : BOOL;
    f7_5 : BOOL;
    f7_6 : BOOL;
    f7_7 : BOOL;
    E_INC1 : BOOL ;     // INC1
    E_INC10 : BOOL ;    // INC10
    E_INC100 : BOOL ;   // INC100
    E_INC1000 : BOOL ;  // INC1000
    E_INC10000 : BOOL ; // INC10000
    E_INCVar : BOOL ;   // INC variable
    f8_6 : BOOL;
    f8_7 : BOOL;
    f9  : BYTE ;
    f10 : ARRAY  [10 .. 19 ] OF BYTE ;
   END_STRUCT ;
  END_STRUCT ;


END_TYPE


//********** MMC-UDT **********
TYPE UDT 19

    STRUCT
   A_SCLight : BOOL ;   //Screen light
   A_SCDark : BOOL ;    //Screen darkening
   A_KeyDisable : BOOL ;      //Key disable
   A_ClearCanAl : BOOL ;      //Clear cancel alarms
   A_ClearRecAl : BOOL ;      //Clear recall alarms
   f0_5 : BOOL ;
   f0_6 : BOOL ;
   A_ActWCS : BOOL ;    //Actual value in WCS 0=MCS
   A_PLCExtViewerReject : BOOL;  //External viewer reject
   A_PLCExtViewerMode   : BOOL;  //External viewer mode
   f1_2                 : BOOL;
   f1_3                 : BOOL;
   f1_4                 : BOOL;
   f1_5                 : BOOL;
   f1_6                 : BOOL;
   f1_7                 : BOOL;
   A_1stError1 : WORD ; //1st error HIGRAPH
   A_1stError2 : WORD ; //1st error HIGRAPH
   A_ASpi1percent : BYTE ;    //Analog spindle 1:
   A_ASpi2percent : BYTE ;
   A_MCPChan : BYTE ;
   A_OEM1 : BOOL ;
   A_OEM2 : BOOL ;
   A_AToolMeas : BOOL ; //AutoToolMeasure
   f9_3 : BOOL ;
   f9_4 : BOOL ;
   f9_5 : BOOL ;
   f9_6 : BOOL ;
   f9_7 : BOOL ;
   A_Hardkey : BYTE ;   //PLC Hardkeys
   f11 : BYTE ;               //Reserved for hardkeys
   f12_0 : BOOL ;
   f12_1 : BOOL ;
   A_COM2 : BOOL ;
   A_COM1 : BOOL ;
   A_V24stop : BOOL ;
   A_V24ext : BOOL ;
   A_V24off : BOOL ;
   A_V24on : BOOL ;
   A_TeachDisable : BOOL ;
   f13_1 : BOOL ;
   f13_2 : BOOL ;
   f13_3 : BOOL ;
   f13_4 : BOOL ;
   A_PPdeload : BOOL ;
   A_PPload : BOOL ;
   A_PPsel : BOOL ;
   A_V24Index1 : BYTE ;
   A_V24Index2 : BYTE ;
   A_V24NoFile1 : BYTE ;
   A_V24NoFile2 : BYTE ;
   A_res18 : BYTE ;
   A_res19 : BYTE ;     //Message counter
   f20_0 : BOOL ;
   E_SCDark : BOOL ;    //Screen darkening
   E_Cancel : BOOL ;    //Cancel
   E_CanCleared : BOOL ;      //Cancel alarms cleared
   E_RecCleared : BOOL ;      //Recall alarms cleared
   f20_5 : BOOL ; //res. Language
   E_SimActiv : BOOL ;  //Simulation active
   E_ActWCS : BOOL ;    //Switchover MCS/WCS 0=MCS
   E_ActivWA : BYTE ;
   E_Chan : BYTE ;      //Channel displayed
   E_KeybHandl    : BOOL;     // Keyboard handling
   E_DataTransf   : BOOL;     // Data transfer active
   E_DisplChange  : BOOL;     // Display change
   f23_3          : BOOL;
   f23_4          : BOOL;
   f23_5          : BOOL;
   f23_6          : BOOL;
   f23_7          : BOOL;
   E_V24Err : BOOL ;
   E_V24OK : BOOL ;
   E_V24COM2 : BOOL ;
   E_V24COM1 : BOOL ;
   E_V24stop : BOOL ;
   E_V24ext : BOOL ;
   E_V24off : BOOL ;
   E_V24on : BOOL ;
   E_V24Error : BYTE ; //V24: Error Byte
   E_res26_0 : BOOL ;     //Reserved
   E_PPOK : BOOL ;     //Part program status OK
   E_PPErr : BOOL ;     //Part program status Error
   E_PPAct : BOOL ;     //Part program status active
   f26_4 : BOOL ;     //Reserved
   E_PPdeload : BOOL ;     //Part program status deloading
   E_PPload : BOOL ;     //Part program status loading
   E_PPsel : BOOL ;     //Part program status selecting
   E_PPError : BYTE ;     //Part program status Error
   A_PictNo : INT ;
   A_PictOn : BOOL ;
   A_PictOff : BOOL ;
   f30_2 : BOOL ;
   f30_3 : BOOL ;
   f30_4 : BOOL ;
   f30_5 : BOOL ;
   f30_6 : BOOL ;
   f30_7 : BOOL ;
   E_PictOK : BOOL ;
   E_PictOn : BOOL ;
   E_PictAct : BOOL ;
   E_PictOff : BOOL ;
   E_PictErr : BOOL ;
   f31_5 : BOOL ;
   f31_6 : BOOL ;
   E_NotAct : BOOL ;
   A_FuncNo : BYTE ;
   A_Par1 : BYTE ;
   A_Par2 : BYTE ;
   A_Par3 : BYTE ;
   E_FuncErr : BYTE ;
   f37 : BYTE;
   f38 : BYTE;
   f39 : BYTE;

   res40 : ARRAY  [0 .. 9 ] OF BYTE  ;
  MMC2: STRUCT
   A_SCLight : BOOL ;   //Screen light
   A_SCDark : BOOL ;    //Screen darkening
   A_KeyDisable : BOOL ;      //Key disable
   A_ClearCanAl : BOOL ;      //Clear cancel alarms
   A_ClearRecAl : BOOL ;      //Clear recall alarms
   f0_5 : BOOL ;
   f0_6 : BOOL ;
   A_ActWCS : BOOL ;    //Actual value in WCS 0=MCS
   A_1stError1 : WORD ; //1st error HIGRAPH
   A_1stError2 : WORD ; //1st error HIGRAPH
   A_ASpi1percent : BYTE ;    //Analog spindle 1:
   A_ASpi2percent : BYTE ;
   A_MCPChan : BYTE ;
   A_OEM1 : BOOL ;
   A_OEM2 : BOOL ;
   A_AToolMeas : BOOL ; //AutoToolMeasure
   f9_3 : BOOL ;
   f9_4 : BOOL ;
   f9_5 : BOOL ;
   f9_6 : BOOL ;
   f9_7 : BOOL ;
   A_Hardkey : BYTE ;   //PLC Hardkeys
   f11 : BYTE ;               //Reserved for hardkeys
   f12_0 : BOOL ;
   f12_1 : BOOL ;
   A_COM2 : BOOL ;
   A_COM1 : BOOL ;
   A_V24stop : BOOL ;
   A_V24ext : BOOL ;
   A_V24off : BOOL ;
   A_V24on : BOOL ;
   f13_0 : BOOL ;
   f13_1 : BOOL ;
   f13_2 : BOOL ;
   f13_3 : BOOL ;
   f13_4 : BOOL ;
   A_PPdeload : BOOL ;
   A_PPload : BOOL ;
   A_PPsel : BOOL ;
   A_V24Index1 : BYTE ;
   A_V24Index2 : BYTE ;
   A_V24NoFile1 : BYTE ;
   A_V24NoFile2 : BYTE ;
   A_res18 : BYTE ;
   A_res19 : BYTE ;     //Message counter
   f20_0 : BOOL ;
   E_SCDark : BOOL ;    //Screen darkening
   E_Cancel : BOOL ;    //Cancel
   E_CanCleared : BOOL ;      //Cancel alarms cleared
   E_RecCleared : BOOL ;      //Recall alarms cleared
   f20_5 : BOOL ; //res. Language
   E_SimActiv : BOOL ;  //Simulation active
   E_ActWCS : BOOL ;    //Switchover MCS/WCS 0=MCS
   E_ActivWA : BYTE ;
   E_Chan : BYTE ;      //Channel displayed
   f23 : BYTE ;
   E_V24Err : BOOL ;
   E_V24OK : BOOL ;
   E_V24COM2 : BOOL ;
   E_V24COM1 : BOOL ;
   E_V24stop : BOOL ;
   E_V24ext : BOOL ;
   E_V24off : BOOL ;
   E_V24on : BOOL ;
   E_V24Error : BYTE ; //V24: Error Byte
   E_res26_0 : BOOL ;     //Reserved
   E_PPOK : BOOL ;     //Part program status OK
   E_PPErr : BOOL ;     //Part program status Error
   E_PPAct : BOOL ;     //Part program status active
   f26_4 : BOOL ;     //Reserved
   E_PPdeload : BOOL ;     //Part program status deloading
   E_PPload : BOOL ;     //Part program status loading
   E_PPsel : BOOL ;     //Part program status selecting
   E_PPError : BYTE ;     //Part program status Error
   A_PictNo : INT ;
   A_PictOn : BOOL ;
   A_PictOff : BOOL ;
   f30_2 : BOOL ;
   f30_3 : BOOL ;
   f30_4 : BOOL ;
   f30_5 : BOOL ;
   f30_6 : BOOL ;
   f30_7 : BOOL ;
   E_PictOK : BOOL ;
   E_PictOn : BOOL ;
   E_PictAct : BOOL ;
   E_PictOff : BOOL ;
   E_PictErr : BOOL ;
   f31_5 : BOOL ;
   f31_6 : BOOL ;
   E_NotAct : BOOL ;
   A_FuncNo : BYTE ;
   A_Par1 : BYTE ;
   A_Par2 : BYTE ;
   A_Par3 : BYTE ;
   E_FuncErr : BYTE ;
   f37 : BYTE;
   f38 : BYTE;
   f39 : BYTE;
   res40 : ARRAY  [0 .. 9 ] OF BYTE  ;
  END_STRUCT ;
//M to N
   ONL_REQUEST : WORD  ;
   ONL_CONFIRM : WORD  ;
   PAR_CLIENT_IDENT : WORD  ;
   PAR_MMC_TYP : BYTE  ;
   PAR_MSTT_ADR : BYTE  ;
   PAR_STATUS : BYTE  ;
   PAR_Z_INFO : BYTE  ;
   MtoNAlive: WORD;
   f112 : Byte;
   ParOpKeyAdr : Byte;
   ParTcuIndex : Byte;
   f115 : Byte  ;
   Tcu1KeyAdr : BYTE  ;
   Tcu2KeyAdr : BYTE  ;
   Tcu1Index : BYTE  ;
   Tcu2Index : BYTE  ;
   MMC1_CLIENT_IDENT : WORD  ;
   MMC1_TYP : BYTE  ;
   MMC1_MSTT_ADR : BYTE  ;
   MMC1_STATUS : BYTE  ;
   MMC1_Z_INFO : BYTE  ;
   MMC1_SHIFT_LOCK : BOOL ;
   MMC1_MSTT_SHIFT_LOCK : BOOL ;
   MMC1_ACTIVE_REQ : BOOL ;
   MMC1_ACTIVE_PERM : BOOL ;
   MMC1_ACTIVE_CHANGED : BOOL ;
   MMC1_CHANGED_DENIED : BOOL ;
   MMC1_TCU_SHIFT_LOCK : BOOL ;
   f127 : BYTE ;
   MMC1_TRANS_DB : Word  ;
   MMC2_CLIENT_IDENT : WORD  ;
   MMC2_TYP : BYTE  ;
   MMC2_MSTT_ADR : BYTE  ;
   MMC2_STATUS : BYTE  ;
   MMC2_Z_INFO : BYTE  ;
   MMC2_SHIFT_LOCK : BOOL ;
   MMC2_MSTT_SHIFT_LOCK : BOOL ;
   MMC2_ACTIVE_REQ : BOOL ;
   MMC2_ACTIVE_PERM : BOOL ;
   MMC2_ACTIVE_CHANGED : BOOL ;
   MMC2_CHANGED_DENIED : BOOL ;
   MMC2_TCU_SHIFT_LOCK : BOOL ;
   f137 : BYTE ;
   MMC2_TRANS_DB : Word ;
   A_Subtype : INT;     //for Codecarrier Input from PLC
   A_Duplo : INT;
   A_Ident : String[32];
   A_Tnumber : INT;
   A_MagazinePlace : INT;
   A_MagazinePlaceType : INT;
   A_ToolSize_Upper : Byte;
   A_ToolSize_Down : Byte;
   A_ToolSize_Left : Byte;
   A_ToolSize_Right : Byte;
   A_Channel : Byte;
   A_LoadingPlace : Byte;
   A_Magazine : INT;
   A_Unit : Byte;
   A_NCU_Index : Byte;
   A_FileIndex : INT;
   A_ActiveEnable : BOOL;
   A_Override : BOOL;
   A_LoadTool : BOOL;
   A_DeleteTool : BOOL;
   //
   E_Subtype : INT;     //for Codecarrier Output to PLC
   E_Duplo : INT;
   E_Ident : String[32];
   E_Tnumber : INT;
   E_ToolState : INT;
   E_MagazinePlaceType : INT;
   E_ToolSize_Upper : Byte;
   E_ToolSize_Down : Byte;
   E_ToolSize_Left : Byte;
   E_ToolSize_Right : Byte;
   E_Magazine : INT;
   E_MagazinePlace : INT;
//
   A_ReqMMC1 : BOOL;  //for Codecarrier Request MMC-Interface1
   A_ReqMMC2 : BOOL;  //for Codecarrier Request MMC-Interface2
   A_K_Code : Byte;
   E_Done : BOOL;
   E_Error : BOOL;
   E_Active : BOOL;
   // CodeCarrierReadEnable : BOOL;
   // CodeCarrierWriteEnable : BOOL;
   E_K_CodeError : Byte; //Identify for Error_Code
   E_Error_Code : INT;

   E_Req : BOOL;  //for Positioning
   f257 : Byte;
   A_Done : BOOL;
   A_Error : BOOL;
   A_Active : BOOL;
   f258_3 : BOOL;
   f258_4 : BOOL;
   f258_5 : BOOL;
   f258_6 : BOOL;
   f258_7 : BOOL;
   E_TDC_Read : BOOL;
   E_TDC_Write : BOOL;
   E_TDC_Cancel : BOOL;
   A_Error_Code : INT;
   E_PMagazine : INT;
   E_PMagazinePlace : INT;
   E_PTnumber : INT;
//TPM-Data
   A_TPMStatus : INT;
   A_TPMCounter : ARRAY [1..32] OF DINT;

   A_HWeelSimOvr : Byte;
   f399 : Byte;
   A_SimOvr : INT;      // simulation overide
   A_SimState : INT;    // simulation state

  END_STRUCT ;


END_TYPE


//********* Channel-UDT *********
TYPE UDT 21

    STRUCT
   f0_0 : BOOL ;
   f0_1 : BOOL ;
   f0_2 : BOOL ;
   A_DRF : BOOL ;   //Activate DRF
   A_SBL : BOOL ;   //Activate single block
   A_M01 : BOOL ;   //Activate M01
   A_DRY : BOOL ;   //Activate dry run feedrate
   f0_7 : BOOL ;
   A_Ref : BOOL ;   //Activate referencing
   A_ProtZone : BOOL ;  //Enable protection zones
   A_SynOff : BOOL ;    //Synchronous action off
   A_TM_TimOut : BOOL ; //Activate time-out (TM)
   A_CLC_Stop : BOOL ;  //CLC stop
   A_CLC_OR : BOOL ;    //CLC override
   A_PLC_ActCompl : BOOL ;  //PLC action complete
   A_ProgTest : BOOL ;  //Activate program test
   A_SKP0 : BOOL ;  //Activate skip block \0
   A_SKP1 : BOOL ;  //Activate skip block \1
   A_SKP2 : BOOL ;  //Activate skip block \2
   A_SKP3 : BOOL ;  //Activate skip block \3
   A_SKP4 : BOOL ;  //Activate skip block \4
   A_SKP5 : BOOL ;  //Activate skip block \5
   A_SKP6 : BOOL ;  //Activate skip block \6
   A_SKP7 : BOOL ;  //Activate skip block \7
   A_StrokEnab : BOOL ; //Stroke enable
   A_ManStrokEnab : BOOL ;  //Manual stroke enable
   A_StrokSup : BOOL ;  //Stroke suppression
   A_StrokDelayed : BOOL ;  //Stroke delayed
   A_StrokStop : BOOL ; //Stroke not operating
   A_ManRelStroke2 : BOOL;      // Manual release of stroke 2
   A3_6 : BOOL;
   A3_7 : BOOL;
   A_FD_OR : BYTE ; //Feedrate override
   A_RT_OR : BYTE ; //Rapid traverse override
   A_FDdisable : BOOL ; //Feed disable
   A_RIdisable : BOOL ; //Read-in disable
   A_DeleteDTG : BOOL ; //Delete distance to go
   A_SP_Clear : BOOL ;  //Clear SP repetitions
   A_ProgAbort : BOOL ; //Program level abort
   A_F_Limit : BOOL ;   //Tool path feedrate limitation
   A_RT_ORA : BOOL ;    //Rapid traverse override active
   A_FD_ORA : BOOL ;    //Feedrate override active
   A_NCStartDisabl : BOOL ; //NC start disable
   A_NCStart : BOOL ;   //NC start
   A_NCStopBlock : BOOL ;   //NC stop at block limit
   A_NCStop : BOOL ;    //NC stop
   A_NCStopASp : BOOL ; //NC stop axes plus spindle
   A_SuppStartLock : BOOL ;   // Suppress Start Lock
   f7_6 : BOOL ;
   A_Reset : BOOL ; //Reset
   A_MRP : ARRAY  [1 .. 10 ] OF BOOL ;  //Activate machine-related protection area [1..10]
   A_CSP : ARRAY  [1 .. 10 ] OF BOOL ;  //Activate channel-specific protection area [1..10]
   A_Geo : ARRAY  [1 .. 3 ] OF STRUCT   //Control signals for geometry axis [1..3]
    HW1 : BOOL ;    //Activate handwheel 1
    HW2 : BOOL ;    //Activate handwheel 2
    HW3 : BOOL ;    //Activate handwheel 3
    FDStop : BOOL ; //Feed stop
    Disabl : BOOL ; //Traversing key disable
    RapidTrOR : BOOL ;  //Rapid traverse override
    Minus : BOOL ;  //Traversing key minus
    Plus : BOOL ;   //Traversing key plus
    INC1 : BOOL ;   //INC 1
    INC10 : BOOL ;  //INC 10
    INC100 : BOOL ; //INC 100
    INC1000 : BOOL ;    //INC 1000
    INC10000 : BOOL ;   //INC 10000
    INCVar : BOOL ; //INC variable
    OEM : BYTE ;    //OEM signals
    InvHWDirOfRot : BOOL;    // Inverting handwheel direction of rotation
    f3_1 : BOOL;
    f3_2 : BOOL;
    f3_3 : BOOL;
    f3_4 : BOOL;
    f3_5 : BOOL;
    f3_6 : BOOL;
    f3_7 : BOOL;
   END_STRUCT ;
   f24_0 : BOOL ;
   f24_1 : BOOL ;
   f24_2 : BOOL ;
   E_MMC_DRF : BOOL ;   //MMC DRF selected
   f24_4 : BOOL ;
   E_MMC_M01 : BOOL ;   //MMC M01 selected
   E_MMC_DRY : BOOL ;   //MMC Dry run feedrate selected
   f24_7 : BOOL ;
   E_MMC_REPOSPM_0 : BOOL ; //MMC REPOSPATHMODE 0
   E_MMC_REPOSPM_1 : BOOL ; //MMC REPOSPATHMODE 1
   E_MMC_REPOSPM_2 : BOOL ; //MMC REPOSPATHMODE 2
   E_MMC_FD_OR4RT_OR : BOOL ;   //MMC Feedrate override for rapid traverse selected
   E_MMC_REPOSMode : BOOL ; //MMC REPOS MODE EDGE
   f25_5 : BOOL ;
   f25_6 : BOOL ;
   E_MMC_ProgTest : BOOL ;  //Program test selected
   E_MMC_SKP0 : BOOL ;  //MMC skip block selected \0
   E_MMC_SKP1 : BOOL ;  //MMC skip block selected \1
   E_MMC_SKP2 : BOOL ;  //MMC skip block selected \2
   E_MMC_SKP3 : BOOL ;  //MMC skip block selected \3
   E_MMC_SKP4 : BOOL ;  //MMC skip block selected \4
   E_MMC_SKP5 : BOOL ;  //MMC skip block selected \5
   E_MMC_SKP6 : BOOL ;  //MMC skip block selected \6
   E_MMC_SKP7 : BOOL ;  //MMC skip block selected \7
   E_MMC_SKP8 : BOOL ;  //MMC skip block selected \8
   E_MMC_SKP9 : BOOL ;  //MMC skip block selected \9
   f27_2 : BOOL ;
   f27_3 : BOOL ;
   f27_4 : BOOL ;
   f27_5 : BOOL ;
   f27_6 : BOOL ;
   f27_7 : BOOL ;
   A_OEM : BYTE ;
   A_FixedFD1 : BOOL ;  //Fixed feeds
   A_FixedFD2 : BOOL ;
   A_FixedFD3 : BOOL ;
   A_FixedFD4 : BOOL ;
   A_PTP_Travel : BOOL ;    //Activate PTP travel
   A_DisablWP_Counter : BOOL ;      //Disable workpiece counter
   A_DisablWearMon : BOOL ; //Disable wear monitoring
   A_DontDisablTool : BOOL ;    //Do not disable tool
   A_ContHW1 : BOOL ;   //Activate contour handwheels
   A_ContHW2 : BOOL ;
   A_ContHW3 : BOOL ;
   A_ContHWsim : BOOL ; //Simulated contour handwheel on
   A_ContHWneg : BOOL ; //Contour handwheel neg. route
   A_NCKrelatedM01 : BOOL ;   // Activate NCK-related M01
   A_JOG_Circles : BOOL ;     // JOG in circles
   A_NoToolChangeCmd : BOOL ; // No tool change commands
   A_REPOSPM_0 : BOOL ; //REPOSPATHMODE 0
   A_REPOSPM_1 : BOOL ; //REPOSPATHMODE 1
   A_REPOSPM_2 : BOOL ; //REPOSPATHMODE 2
   f31_3 : BOOL ;
   A_REPOSMode : BOOL ; //REPOS MODE EDGE
   A_InvCHWDirOfRot : BOOL;      // Inverting contour handwheel direction of rotation
   A_SKP8 : BOOL ;  //Activate skip block \8
   A_SKP9 : BOOL ;  //Activate skip block \9
   E_ExecExtern : BOOL ;//Execution from external source active
   f32_1 : BOOL ;
   f32_2 : BOOL ;
   E_ActBlock : BOOL ;  //Action block active
   E_BegBlock : BOOL ;  //Approach block active
   E_M01 : BOOL ;   //M0/M1 active
   E_LastActBlock : BOOL ;  //Last action block active
   f32_7 : BOOL ;
   E_Ref : BOOL ;   //Referencing active
   E_OrieToolholder : BOOL ;  // Orientable toolholder active
   E_RevFD : BOOL ; //Revolutional feedrate active
   E_HWOverlay : BOOL ; //Handwheel overlay active
   E_BlockSearch : BOOL ;   //Block search active
   E_M30 : BOOL ;   //M2/M30 active
   E_Transform : BOOL ; //Transformation active
   E_ProgTest : BOOL ;  //Program test active
   E_OEMChan : BYTE ;   //OEM channel signals feedback
   E_ProgRunn : BOOL ;  //Program running
   E_ProgWait : BOOL ;  //Program waiting
   E_ProgStop : BOOL ;  //Program stopped
   E_ProgInterrupt : BOOL ; //Program interrupted
   E_ProgrAborted : BOOL ;  //Program aborted
   E_ChanActive : BOOL ;    //Channel active
   E_ChanInterrupt : BOOL ; //Channel interrupted
   E_ChanReset : BOOL ; //Channel reset
   E_StartReq : BOOL ;  //Start request
   E_StopReq : BOOL ;   //Stop request
   E_AxesRef : BOOL ;   //All axes referenced
   E_AxesStop : BOOL ;  //All axes stationary
   E_IR_Activ : BOOL ;  //Interrupt processing active
   E_ChanRO : BOOL ;    //Channel ready for operation
   E_NCKalarmChan : BOOL ;  //Channel-specific NCK alarm present
   E_NCKalarmStop : BOOL ;  //NCK alarm with processing stop present
   E_CHW1 : BOOL ;  //Contour handwheel 1 on
   E_CHW2 : BOOL ;  //Contour handwheel 2 on
   E_CHW3 : BOOL ;  //Contour handwheel 3 on
   E_CLC : BOOL ;   //CLC active
   E_CLCStopLL : BOOL ; //CLC stopped lower limit
   E_CLCStopUL : BOOL ; //CLC stopped upper limit
   E_RIEnabIgnored : BOOL ; //Read-in enable is ignored
   E_StopBlkEndSBLsuppr : BOOL ;    //Stop at block end with SBL is suppressed
   E_StrokeEA : BOOL ;  //Stroke enable active
   E_AcknManStrokEnab : BOOL ;  //Acknowledgement manual stroke enable
   f38_2 : BOOL ;
   f38_3 : BOOL ;
   f38_4 : BOOL ;
   f38_5 : BOOL ;
   f38_6 : BOOL ;
   f38_7 : BOOL ;
   E_ProtZoneNOK : BOOL ;   //Protection zones not guaranteed
   f39_1 : BOOL;
   f39_2 : BOOL;
   f39_3 : BOOL;
   f39_4 : BOOL;
   E_InvCHWDirOfRot : BOOL;      // Contour handwheel direction of rotation invert actively
   f39_6 : BOOL;
   f39_7 : BOOL;
   E_Geo : ARRAY  [1 .. 3 ] OF STRUCT   //Status signals of geometry axis [1..3]
    HW1 : BOOL ;    //Handwheel 1 active
    HW2 : BOOL ;    //Handwheel 2 active
    HW3 : BOOL ;    //Handwheel 3 active
    f0_3 : BOOL ;
    TReqMinus : BOOL ;  // Travel requests minus
    TReqPlus : BOOL ;   // Travel requests plus
    TCMinus : BOOL ;    //Traverse command minus
    TCPlus : BOOL ; //Traverse command plus
    INC1 : BOOL ;   //INC 1 active
    INC10 : BOOL ;  //INC 10 active
    INC100 : BOOL ; //INC 100 active
    INC1000 : BOOL ;    //INC 1000 active
    INC10000 : BOOL ;   //INC 10000 active
    INCVar : BOOL ; //INC variable active
    OEM : BYTE ;    //OEM signals
    InvHWDirOfRot : BOOL;     // Handwheel direction of rotation invert actively
    f3_1 : BOOL;
    f3_2 : BOOL;
    f3_3 : BOOL;
    f3_4 : BOOL;
    f3_5 : BOOL;
    f3_6 : BOOL;
    f3_7 : BOOL;
    f4 : BYTE;
   END_STRUCT ;
   M1Change : BOOL ;    //M function 1 change
   M2Change : BOOL ;    //M function 2 change
   M3Change : BOOL ;    //M function 3 change
   M4Change : BOOL ;    //M function 4 change
   M5Change : BOOL ;    //M function 5 change
   f58_5 : BOOL ;
   f58_6 : BOOL ;
   f58_7 : BOOL ;
   M1NDec : BOOL ;  //M function 1 not decoded
   M2NDec : BOOL ;  //M function 2 not decoded
   M3NDec : BOOL ;  //M function 3 not decoded
   M4NDec : BOOL ;  //M function 4 not decoded
   M5NDec : BOOL ;  //M function 5 not decoded
   f59_5 : BOOL ;
   f59_6 : BOOL ;
   f59_7 : BOOL ;
   S1Change : BOOL ;    //S function 1 change
   S2Change : BOOL ;    //S function 2 change
   S3Change : BOOL ;    //S function 3 change
   f60_3 : BOOL ;
   S1Quick : BOOL ; //S function 1 quick
   S2Quick : BOOL ; //S function 2 quick
   S3Quick : BOOL ; //S function 3 quick
   f60_7 : BOOL ;
   T1Change : BOOL ;    //T function 1 change
   T2Change : BOOL ;    //T function 2 change
   T3Change : BOOL ;    //T function 3 change
   f61_3 : BOOL ;
   T1Quick : BOOL ; //T function 1 quick
   T2Quick : BOOL ; //T function 2 quick
   T3Quick : BOOL ; //T function 3 quick
   f61_7 : BOOL ;
   D1Change : BOOL ;    //D function 1 change
   D2Change : BOOL ;    //D function 2 change
   D3Change : BOOL ;    //D function 3 change
   f62_3 : BOOL ;
   D1Quick : BOOL ; //D function 1 quick
   D2Quick : BOOL ; //D function 2 quick
   D3Quick : BOOL ; //D function 3 quick
   f62_7 : BOOL ;
   EChange : BOOL ; //E function change
   f63_1 : BOOL ;
   f63_2 : BOOL ;
   f63_3 : BOOL ;
   EQuick : BOOL ;  //E function quick
   f63_5 : BOOL ;
   f63_6 : BOOL ;
   f63_7 : BOOL ;
   H1Change : BOOL ;    //H function 1 change
   H2Change : BOOL ;    //H function 2 change
   H3Change : BOOL ;    //H function 3 change
   f64_3 : BOOL ;
   H1Quick : BOOL ; //H function 1 quick
   H2Quick : BOOL ; //H function 2 quick
   H3Quick : BOOL ; //H function 3 quick
   f64_7 : BOOL ;
   F1Change : BOOL ;    //F function 1 change
   F2Change : BOOL ;    //F function 2 change
   F3Change : BOOL ;    //F function 3 change
   F4Change : BOOL ;    //F function 4 change
   F5Change : BOOL ;    //F function 5 change
   F6Change : BOOL ;    //F function 6 change
   f65_6 : BOOL ;
   f65_7 : BOOL ;
   M1Quick : BOOL ; //M function 1 quick
   M2Quick : BOOL ; //M function 2 quick
   M3Quick : BOOL ; //M function 3 quick
   M4Quick : BOOL ; //M function 4 quick
   M5Quick : BOOL ; //M function 5 quick
   f66_5 : BOOL ;
   f66_6 : BOOL ;
   f66_7 : BOOL ;
   F1Quick : BOOL ; //F function 1 quick
   F2Quick : BOOL ; //F function 2 quick
   F3Quick : BOOL ; //F function 3 quick
   F4Quick : BOOL ; //F function 4 quick
   F5Quick : BOOL ; //F function 5 quick
   F6Quick : BOOL ; //F function 6 quick
   f67_6 : BOOL ;
   f67_7 : BOOL ;
   ExtM1 : INT ;    //Extended address M function 1 (16 bit INT)
   M1 : DINT ;  //M function 1 (DInt)
   ExtM2 : INT ;    //Extended address M function 1 (16 bit INT)
   M2 : DINT ;  //M function 2 (DInt)
   ExtM3 : INT ;    //Extended address M function 1 (16 bit INT)
   M3 : DINT ;  //M function 3 (DInt)
   ExtM4 : INT ;    //Extended address M function 1 (16 bit INT)
   M4 : DINT ;  //M function 4 (DInt)
   ExtM5 : INT ;    //Extended address M function 1 (16 bit INT)
   M5 : DINT ;  //M function 5 (DInt)
   ExtS1 : INT ;    //Extended address S function 1 (16 bit INT)
   S1 : REAL ;  //S function 1 (REAL)
   ExtS2 : INT ;    //Extended address S function 2 (16 bit INT)
   S2 : REAL ;  //S function 2 (REAL)
   ExtS3 : INT ;    //Extended address S function 3 (16 bit INT)
   S3 : REAL ;  //S function 3 (REAL)
   ExtT1 : INT ;    //Extended address T function 1 (16 bit INT)
//T : DINT; //T function (DInt)
//f122 : INT;
//f124 : INT;
//f126 : INT;   //Change in case of 8-digit T function

   T1 : INT ;   //T function 1 (INT)
   ExtT2 : INT ;    //Extended address T function 2 (16 bit INT)
   T2 : INT ;   //T function 2 (INT)
   ExtT3 : INT ;    //Extended address T function 3 (16 bit INT)
   T3 : INT ;   //T function 3 (INT)
   ExtD1 : BYTE ;   //Extended address D function 1 (8 bit INT)
//D : INT;
//f132 : INT;   //Change in case of 5-digit D function

   D1 : BYTE ;  //D function 1 (8 bit INT)
   ExtD2 : BYTE ;   //Extended address D function 2 (8 bit INT)
   D2 : BYTE ;  //D function 2 (8 bit INT)
   ExtD3 : BYTE ;   //Extended address D function 3 (8 bit INT)
   D3 : BYTE ;  //D function 3 (8 bit INT)
   ExtE : INT ; //Extended address E function 3 (16 bit INT)
   E : REAL ;   //E function (REAL)
   ExtH1 : INT ;    //Extended address H function 1 (16 bit INT)
   H1 : REAL ;  //H function 1 (REAL)
   ExtH2 : INT ;    //Extended address H function 2 (16 bit INT)
   H2 : REAL ;  //H function 2 (REAL)
   ExtH3 : INT ;    //Extended address H function 3 (16 bit INT)
   H3 : REAL ;  //H function 3 (REAL)
   ExtF1 : INT ;    //Extended address F function 1 (16 bit INT)
   F1 : REAL ;  //F function 1 (REAL)
   ExtF2 : INT ;    //Extended address F function 2 (16 bit INT)
   F2 : REAL ;  //F function 2 (REAL)
   ExtF3 : INT ;    //Extended address F function 3 (16 bit INT)
   F3 : REAL ;  //F function 3 (REAL)
   ExtF4 : INT ;    //Extended address F function 4 (16 bit INT)
   F4 : REAL ;  //F function 4 (REAL)
   ExtF5 : INT ;    //Extended address F function 5 (16 bit INT)
   F5 : REAL ;  //F function 5 (REAL)
   ExtF6 : INT ;    //Extended address F function 6 (16 bit INT)
   F6 : REAL ;  //F function 6 (REAL)
   MDyn : ARRAY  [0 .. 99 ] OF BOOL ;   //Dynamic M functions [0..99]
   GAct : ARRAY  [1 .. 64 ] OF BYTE ;   //Active G function of group [1..64]
   E_MRPactivated : ARRAY  [1 .. 10 ] OF BOOL ; //Machine-related protection area [1..10] preactivated
   E_CSPactivated : ARRAY  [1 .. 10 ] OF BOOL ; //Channel-specific protection area [1..10] preactivated
   E_MRPViolated : ARRAY  [1 .. 10 ] OF BOOL ;  //Machine-related protection area [1..10] violated
   E_CSPViolated : ARRAY  [1 .. 10 ] OF BOOL ;  //Channel-specific protection area [1..10] violated
//from P4 on
   A_Str_DNo : BOOL ;   //Request of D number to NCK
   A_Str_Synon : BOOL ; //Request of syn.action to NCK
   f_280_2 : BOOL ;
   f_280_3 : BOOL ;
   f_280_4 : BOOL ;
   f_280_5 : BOOL ;
   f_280_6 : BOOL ;
   f_280_7 : BOOL ;
   f_281_0 : BOOL ;
   A_Str_Synfrom : BOOL ;   //Request syn.action from NCK
   f_281_2 : BOOL ;
   f_281_3 : BOOL ;
   f_281_4 : BOOL ;
   f_281_5 : BOOL ;
   f_281_6 : BOOL ;
   f_281_7 : BOOL ;
   A_D1 : INT ; //Assignment D1
   A_D2 : INT ; //Assignment D2
   A_D3 : INT ; //Assignment D3
   A_D4 : INT ; //Assignment D4
   A_D5 : INT ; //Assignment D5
   A_D6 : INT ; //Assignment D6
   A_D7 : INT ; //Assignment D7
   A_D8 : INT ; //Assignment D8
   A_D9 : INT ; //Assignment D9
   A_SynDisabl : ARRAY  [1 .. 64 ] OF BOOL ;    //Disable synchronous actions
   E_SynDisabled : ARRAY  [1 .. 64 ] OF BOOL ;  //Synchronous actions disabled
   E_G00 : BOOL ;             //Active G functions
   f316_1 : BOOL ;
   f316_2 : BOOL ;
   f316_3 : BOOL ;
   f316_4 : BOOL ;
   f316_5 : BOOL ;
   f316_6 : BOOL ;
   f316_7 : BOOL ;
   E_ExtLang : BOOL ;         // External language mode active
   E_WS_Setp : BOOL ;         // Workpiece setpoint reached
   f317_2 : BOOL ;
   f317_3 : BOOL ;
   f317_4 : BOOL ;
   E_DriveTest : BOOL ;       // Travel request drive test
   E_PTP_Travel : BOOL ;      //PTP travel active
   E_ToolMissing : BOOL ;     //Tool missing
   E_ASUP_Stop : BOOL;        // ASUP stopped
   E_SearchAct : BOOL;        // Search active
   E_TOFF : BOOL;             // TOFF active
   E_TOFFmovem : BOOL;        // TOFF movement active
   E_StopDelayed : BOOL;      // Stop delayed
   E_AssM01 : BOOL;           // Associated M01 active
   E_DRY : BOOL;              // Dry-run feedrate active
   E_Overstore : BOOL;        // Overstore active
   E_REPOS_EdgeAckn : BOOL;   // REPOS MODE EDGE ACKN
   E_REPOS_PMode0 : BOOL;     // Repos Path Mode Ackn 0
   E_REPOS_PMode1 : BOOL;     // Repos Path Mode Ackn 0
   E_REPOS_PMode2 : BOOL;     // Repos Path Mode Ackn 2
   E_DelayFTS : BOOL;         // Delay FTS
   E_REPOS_DEFERRA : BOOL;    // Repos DEFERRA L Chan
   E_Stop_NoDelayR : BOOL;    // Stop-delayrange not activated
   E_NoToolChangeCmd : BOOL;  // No tool change command active
  A_Ori : ARRAY  [1 .. 3 ] OF STRUCT    //Control signals for orientation axes [1..3]
    HW_Bit0 : BOOL ;    //Activate handwheel Bit value coding
    HW_Bit1 : BOOL ;    //Activate handwheel Bit value coding
    HW_Bit2 : BOOL ;    //Activate handwheel Bit value coding
    FDStop : BOOL ; //Feed stop
    Disabl : BOOL ; //Traversing key disable
    RapidTrOR : BOOL ;  //Rapid traverse override
    Minus : BOOL ;  //Traversing key minus
    Plus : BOOL ;   //Traversing key plus
    INC1 : BOOL ;   //INC 1 active
    INC10 : BOOL ;  //INC 10 active
    INC100 : BOOL ; //INC 100 active
    INC1000 : BOOL ;    //INC 1000 active
    INC10000 : BOOL ;   //INC 10000 active
    INCVar : BOOL ; //INC variable active
    OEM : BYTE ;    //OEM signals
    InvHWDirOfRot : BOOL;     // Inverting handwheel direction of rotation
    f3_1 : BOOL;
    f3_2 : BOOL;
    f3_3 : BOOL;
    f3_4 : BOOL;
    f3_5 : BOOL;
    f3_6 : BOOL;
    f3_7 : BOOL;
   END_STRUCT ;
  E_Ori : ARRAY  [1 .. 3 ] OF STRUCT    //Control signals for orientation axes [1..3]
    HW_Bit0 : BOOL ;    //Activate handwheel Bit value coding
    HW_Bit1 : BOOL ;    //Activate handwheel Bit value coding
    HW_Bit2 : BOOL ;    //Activate handwheel Bit value coding
    f0_3 : BOOL ;
    TReqMinus : BOOL ;  // Travel requests minus
    TReqPlus : BOOL ;   // Travel requests plus
    Minus : BOOL ;  //Traversing key minus
    Plus : BOOL ;   //Traversing key plus
    INC1 : BOOL ;   //INC 1 active
    INC10 : BOOL ;  //INC 10 active
    INC100 : BOOL ; //INC 100 active
    INC1000 : BOOL ;    //INC 1000 active
    INC10000 : BOOL ;   //INC 10000 active
    INCVar : BOOL ; //INC variable active
    OEM : BYTE ;    //OEM signals
    InvHWDirOfRot : BOOL;     // Handwheel direction of rotation invert actively
    f3_1 : BOOL;
    f3_2 : BOOL;
    f3_3 : BOOL;
    f3_4 : BOOL;
    f3_5 : BOOL;
    f3_6 : BOOL;
    f3_7 : BOOL;
   END_STRUCT ;
   E_T_PrewarnLimit : BOOL ;    //Tool prewarn limit reached
   E_T_Limit : BOOL ;   //Tool limit reached
   E_NewReplT : BOOL ;  //Transition to new replacement tool
   E_LastReplT : BOOL ; //last replacement tool of the tool group
   f344_4 : BOOL;
   f344_5 : BOOL;
   f344_6 : BOOL;
   f344_7 : BOOL;
   f345 : BYTE ;
   f346 : BYTE ;
   f347 : BYTE ;
   E_T_NoPrewarnLimit : DINT ;  //T number for tool prewarn limit
   E_T_NoLimit : DINT ; //T number for tool limit
   E_NewReplT_No : DINT ;   //T number of the new replacement tool
   E_LastReplT_No : DINT ;  //T number of the last replacement tool
   E_Cycle_Sig : ARRAY  [0 .. 15 ] OF BOOL ;  //Cycles Input Signals
   A_Cycle_Sig : ARRAY  [0 .. 15 ] OF BOOL ;  //Cycles Output Signals
   E_OEM_TechnoSig : ARRAY  [0 .. 31 ] OF BOOL ;  //OEM Techno Input Signals
   A_OEM_TechnoSig : ARRAY  [0 .. 31 ] OF BOOL ;  //OEM Techno Output Signals
   ProgEventDispl       : BYTE ;    // ProgEventDisplay
   E_CollCheckStop      : BOOL;     // Stop of Collision Check
   E_StopCondition      : BOOL ;    // Stop Condition
   f377_2 : BOOL ;
   f377_3 : BOOL ;
   E_JogRetract : BOOL ;      // JOG Retract active
   E_RetractData : BOOL ;     // Retract data available
   E_JOG_Circles : BOOL ;     // JOG in circles
   f377_7 : BOOL ;
   E_AnyAsup : BOOL ;         // AnyASUP activ
   E_SilentAsup : BOOL ;      // Silent ASUP activ
   f378_2 : BOOL ;
   f378_3 : BOOL ;
   f378_4 : BOOL ;
   f378_5 : BOOL ;
   f378_6 : BOOL ;
   f378_7 : BOOL ;
   f379 : BYTE ;
   f380 : ARRAY  [0 .. 31 ] OF BOOL ;  //Reserved
   A_ProgJump : BOOL;         // control program jump
   f384_1 : BOOL;
   f384_2 : BOOL;
   f384_3 : BOOL;
   f384_4 : BOOL;
   f384_5 : BOOL;
   f384_6 : BOOL;
   f384_7 : BOOL;
   A_InKeyG1        : BOOL;     // Grinding signal 1
   A_InKeyG2        : BOOL;     // Grinding signal 2
   A_InKeyG3        : BOOL;     // Grinding signal 3
   A_InKeyG4        : BOOL;     // Grinding signal 4
   A_InKeyG5        : BOOL;     // Grinding signal 5
   A_InKeyG6        : BOOL;     // Grinding signal 6
   A_InKeyG7        : BOOL;     // Grinding signal 7
   A_InKeyG8        : BOOL;     // Grinding signal 8
   A_InKeyGEn1      : BOOL;     // Enable grinding signal 1
   A_InKeyGEn2      : BOOL;     // Enable grinding signal 2
   A_InKeyGEn3      : BOOL;     // Enable grinding signal 3
   A_InKeyGEn4      : BOOL;     // Enable grinding signal 4
   A_InKeyGEn5      : BOOL;     // Enable grinding signal 5
   A_InKeyGEn6      : BOOL;     // Enable grinding signal 6
   A_InKeyGEn7      : BOOL;     // Enable grinding signal 7
   A_InKeyGEn8      : BOOL;     // Enable grinding signal 8
   A_InKeyGRunIn1   : BOOL;     // Run grinding function 1
   A_InKeyGRunIn2   : BOOL;     // Run grinding function 2
   A_InKeyGRunIn3   : BOOL;     // Run grinding function 3
   A_InKeyGRunIn4   : BOOL;     // Run grinding function 4
   A_InKeyGRunIn5   : BOOL;     // Run grinding function 5
   A_InKeyGRunIn6   : BOOL;     // Run grinding function 6
   A_InKeyGRunIn7   : BOOL;     // Run grinding function 7
   A_InKeyGRunIn8   : BOOL;     // Run grinding function 8
   E_TransfoNo : BYTE;          // active transformation number
   f389        : BYTE;
   E_InKeyGIsEn1    : BOOL;     // Grinding signal 1 enabled
   E_InKeyGIsEn2    : BOOL;     // Grinding signal 2 enabled
   E_InKeyGIsEn3    : BOOL;     // Grinding signal 3 enabled
   E_InKeyGIsEn4    : BOOL;     // Grinding signal 4 enabled
   E_InKeyGIsEn5    : BOOL;     // Grinding signal 5 enabled
   E_InKeyGIsEn6    : BOOL;     // Grinding signal 6 enabled
   E_InKeyGIsEn7    : BOOL;     // Grinding signal 7 enabled
   E_InKeyGIsEn8    : BOOL;     // Grinding signal 8 enabled
   E_InKeyGRunOut1  : BOOL;     // NCK status of grinding function 1
   E_InKeyGRunOut2  : BOOL;     // NCK status of grinding function 3
   E_InKeyGRunOut3  : BOOL;     // NCK status of grinding function 3
   E_InKeyGRunOut4  : BOOL;     // NCK status of grinding function 4
   E_InKeyGRunOut5  : BOOL;     // NCK status of grinding function 5
   E_InKeyGRunOut6  : BOOL;     // NCK status of grinding function 6
   E_InKeyGRunOut7  : BOOL;     // NCK status of grinding function 7
   E_InKeyGRunOut8  : BOOL;     // NCK status of grinding function 8
   E_CART_JOG_MODE  : BYTE;     // Coordinate system for Cartesian jog traverse
   f393             : BYTE;
   f394             : BYTE;
   f395             : BYTE;
  END_STRUCT ;


END_TYPE


//***** Axis-/Spindle-UDT *****
TYPE UDT 31


  STRUCT
   A_FD_OR : BYTE ; //Feedrate override
   A_DriveEnable : BOOL ;   //Drive test movement enable
   A_AckFixedStop : BOOL ;  //Acknowledge fixed stop reached
   A_SensorFixedStop : BOOL ;   //Sensor fixed stop
   A_ASpDisable : BOOL ;    //Axis/spindle disable
   A_Follow_upMode : BOOL ; //Follow-up mode
   A_PosMeas1 : BOOL ;  //Position measuring system 1
   A_PosMeas2 : BOOL ;  //Position measuring system 2
   A_ORactive : BOOL ;  //Override active
   A_SWCam : BOOL ; //SW cam activation
   A_ContrEnable : BOOL ;   //Controller enable
   A_DelDTGSpReset : BOOL ; //Delete distance to go/Spindle-Reset
   A_Clamp : BOOL ; //Clamping in progress
   A_RefVal1 : BOOL ;   //Reference point value 1
   A_RefVal2 : BOOL ;   //Reference point value 2
   A_RefVal3 : BOOL ;   //Reference point value 3
   A_RefVal4 : BOOL ;   //Reference point value 4
   A_ExtZO : BOOL ; //Import external ZO
   A_EnabTravFixedStop : BOOL ; //Enable travel to fixed stop
   A_FixedFD1 : BOOL ;  //Activate fixed feed 1
   A_FixedFD2 : BOOL ;  //Activate fixed feed 2
   A_FixedFD3 : BOOL ;  //Activate fixed feed 3
   A_FixedFD4 : BOOL ;  //Activate fixed feed 4
   A_VelocSpeedLimit : BOOL ;   //Velocity/spindle speed limitation
   A_PrgtestAxRel : BOOL ;    // Program test axis/spindle release
   A_HW1 : BOOL ;   //Activate handwheel 1
   A_HW2 : BOOL ;   //Activate handwheel 2
   A_HW3 : BOOL ;   //Activate handwheel 3
   A_FDSpStop : BOOL ;  //Feed stop/spindle stop
   A_Disable : BOOL ;   //Traversing key disable
   A_RapidTrOR : BOOL ; //Rapid traverse override
   A_Minus : BOOL ; //Traversing key minus
   A_Plus : BOOL ;  //Traversing key plus
   A_INC1 : BOOL ;  //INC1
   A_INC10 : BOOL ; //INC10
   A_INC100 : BOOL ;    //INC100
   A_INC1000 : BOOL ;   //INC1000
   A_INC10000 : BOOL ;  //INC10000
   A_INCVar : BOOL ;    //INC variable
   A_OEMAxis : BYTE ;   //OEM axis signals
   A_InvHWDirOfRot : BOOL;    // Inverting handwheel direction of rotation
   f7_1  : BOOL;
   f7_2  : BOOL;
   f7_3  : BOOL;
   f7_4  : BOOL;
   f7_5  : BOOL;
   f7_6  : BOOL;
   f7_7  : BOOL;
   A_NCASpChanA : BOOL ;    //Assign NC axis/spindle channel A
   A_NCASpChanB : BOOL ;    //Assign NC axis/spindle channel B
   A_NCASpChanC : BOOL ;    //Assign NC axis/spindle channel C
   A_NCASpChanD : BOOL ;    //Assign NC axis/spindle channel D
   A_NCASpStrobe : BOOL ;   //Activation of assignment with pos. edge
   f8_5 : BOOL ;
   f8_6 : BOOL ;
   A_PLCASp : BOOL ;    //Request PLC axis/spindle
   A_Para_A : BOOL ;    //Parameter block servo A
   A_Para_B : BOOL ;    //Parameter block servo B
   A_Para_C : BOOL ;    //Parameter block servo C
   A_LockParSetDef : BOOL ; //Lock parameter set definition from NC
   f9_4 : BOOL ;
   f9_5 : BOOL ;
   f9_6 : BOOL ;
   f9_7 : BOOL ;
   A_REPOSDelay : BOOL ;    //REPOS DELAY
   f10_1 : BOOL ;
   f10_2 : BOOL ;
   f10_3 : BOOL ;
   f10_4 : BOOL ;
   f10_5 : BOOL ;
   f10_6 : BOOL ;
   f10_7 : BOOL ;
   A_StartBrakeTest : BOOL;   // Start brake test
   f11_1 : BOOL;
   f11_2 : BOOL;
   f11_3 : BOOL;
   f11_4 : BOOL;
   f11_5 : BOOL;
   f11_6 : BOOL;
   f11_7 : BOOL;
   A_HWLimitMinus : BOOL ;  //Hardware limit switch minus
   A_HWLimitPlus : BOOL ;   //Hardware limit switch plus
   A_SWLimit2Minus : BOOL ; //2nd software limit switch minus
   A_SWLimit2Plus : BOOL ;  //2nd software limit switch plus
   A_ModuloLimitEn : BOOL ;   // Modulo limit enabled
   f12_5 : BOOL ;
   f12_6 : BOOL ;
   A_DelayRef : BOOL ;        //Delay reference point approach
   A_JogFixPPos0  : BOOL;     // JogFixPointPos 0
   A_JogFixPPos1  : BOOL;     // JogFixPointPos 1
   A_JogFixPPos2  : BOOL;     // JogFixPointPos 2
   A_JogToPos : BOOL;         // Jog to position
   f13_4 : BOOL;
   f13_5 : BOOL;
   f13_6 : BOOL;
   f13_7 : BOOL;


   A_ProgtestSuppress   : BOOL;  // Program test to supress
   A_ProgtestActivate   : BOOL;  // Program test activate
   f14_2                : BOOL;
   f14_3                : BOOL;
   f14_4                : BOOL;
   f14_5                : BOOL;
   f14_6                : BOOL;
   f14_7                : BOOL;
   f15                  : BYTE;

   A_ActGearA : BOOL ;  //Actual gear stage A
   A_ActGearB : BOOL ;  //Actual gear stage B
   A_ActGearC : BOOL ;  //Actual gear stage C
   A_GearChangeOv : BOOL ;  //Gear has changed over
   A_Sp1Syn : BOOL ;    //Re-synchronize spindle 1
   A_Sp2Syn : BOOL ;    //Re-synchronize spindle 2
   A_NoMonitorGear : BOOL ; //No monitoring when changing gear
   A_DeleteS : BOOL ;   //Delete S value
   A_FD_ORSp : BOOL ;   //Feedrate override for spindle valid
   f17_1 : BOOL ;
   f17_2 : BOOL ;
   f17_3 : BOOL ;
   A_Sp1SynP : BOOL ;   //Re-synchronize spindle 1 f. positioning
   A_Sp2SynP : BOOL ;   //Re-synchronize spindle 2 f. positioning
   A_M3M4Inv : BOOL ;   //Invert M3/M4
   f17_7 : BOOL ;
   f18_0 : BOOL ;
   f18_1 : BOOL ;
   f18_2 : BOOL ;
   f18_3 : BOOL ;
   A_OscilPLC : BOOL ;  //Oscillation via PLC
   A_OscilSpeed : BOOL ;    //enable Oscillation
   A_SetRotDirectRight : BOOL ; //Setpoint osci. direct. right
   A_SetRotDirectLeft : BOOL ;  //Setpoint osci. direct. left
   A_SpOR : BYTE ;  //Spindle override
   f20_0 : BOOL ;
   A_RUEncQuStop : BOOL ;   //Run-up encoder quick stop
   f20_2 : BOOL ;
   A_SpeedSetpSmooth : BOOL ;   //Speed setpoint smoothing
   f20_4 : BOOL ;
   A_HoldBrakeToOpen : BOOL ;   // holding brake open
   f20_6 : BOOL ;
   f20_7 : BOOL ;
   A_ParA : BOOL ;  //Parameter set selection A
   A_ParB : BOOL ;  //Parameter set selection B
   A_ParC : BOOL ;  //Parameter set selection C
   A_MotA : BOOL ;  //Motor selection A
   A_MotB : BOOL ;  //Motor selection B
   A_MotOK : BOOL ; //Motor selected
   A_IntegratDisable : BOOL ;   //n controller integrator disable
   A_PulseEnable : BOOL ;   //Pulse enable

   A_SG_SBH : BOOL ;         //Deselection SG/SBH
   A_SBH : BOOL ;                //Deselection of safe standstill
   f22_2 : BOOL ;
   A_SGselect0 : BOOL ;          //Selection SG bit 0
   A_SGselect1 : BOOL ;          //Selection SG bit 1
   f22_5 : BOOL ;
   f22_6 : BOOL ;
   f22_7 : BOOL ;
   A_Transmiss0 : BOOL ;         //Selection Transmission bit 0
   A_Transmiss1 : BOOL ;         //Selection Transmission bit 1
   A_Transmiss2 : BOOL ;         //Selection Transmission bit 2
   f23_3 : BOOL ;
   A_SE : BOOL ;                   //Selection SE
   A_BrakeToClose : BOOL ;       //Sinamics: Brake to close
   f23_6 : BOOL ;
   A_TestStop : BOOL ;           //Activate test stop

   A_RotationMonit : BOOL ;   // Stepper motor: Rotation monitoring
   A_ControlAx : BOOL ;       // Control Axis
   f24_2 : BOOL ;
   f24_3 : BOOL ;
   A_TorqComp : BOOL;               // Torque compensation
   A_ChangSetpOutAss0 : BOOL ;      // Bit value for CTRLOUT_changed - Change setpoint output assignment
   A_ChangSetpOutAss1 : BOOL ;      // Bit value for CTRLOUT_changed - Change setpoint output assignment
   A_MS : BOOL ;                    //Master / Slave On
   A_DynBComp : BOOL;   // dynamic backlash compensation activated
   f25_1 : BOOL ;
   f25_2 : BOOL ;
   f25_3 : BOOL ;
   f25_4 : BOOL ;
   f25_5 : BOOL ;
   f25_6 : BOOL ;
   f25_7 : BOOL ;
   f26_0 : BOOL ;
   f26_1 : BOOL ;
   f26_2 : BOOL ;
   A_CompContr : BOOL ; //Compensation controller On
   A_FollowAxOv : BOOL ;    //Enable following axis override
   f26_5 : BOOL ;
   f26_6 : BOOL ;
   f26_7 : BOOL ;
   A_DEPMCS : BOOL;           // Resume: DEPMCS
   A_DEPBCS : BOOL;           // Resume: DEPBCS
   A_Corr : BOOL;             // Resume: Corr
   A_HIAxMove : BOOL;         // Resume: HIAxMove
   A_StopDEPMCS : BOOL;     // Stop: DEPMCS
   A_StopDEPBCS : BOOL;     // Stop: DEPBCS
   A_StopCorr : BOOL;       // Stop: Corr
   A_StopHIAxMove : BOOL;   // Stop: HIAxMove
   A_OscillAxExtRev : BOOL ;  // OscillAxExtReversal
   A_AxReset : BOOL ;         // AXRESET
   A_AxResume : BOOL ;        // AXRESUME
   A_SetRP : BOOL ; //Set reversal point
   A_ChangeRP : BOOL ;  //Change reversal point
   A_StopRP : BOOL ;    //Stop at next reversal point
   A_Stop : BOOL ;  //Stop
   A_PLCAxis : BOOL ;   //PLC checks axis
   f29_0 : BOOL ;
   f29_1 : BOOL ;
   f29_2 : BOOL ;
   f29_3 : BOOL ;
   A_StartGantSynRun : BOOL ;   //Start gantry synchronization run
   A_NoAutoSync : BOOL ;    //No auto sync
   f29_6 : BOOL ;
   f29_7 : BOOL ;
   A_StopSpindle : BOOL ;   //Stop spindle
   A_StartCW : BOOL ;   //Start spindle Clockwise
   A_StartCCW : BOOL ;  //Start spindle Counterclockwise
   A_AutoGearStep : BOOL ;  //Autom. gear step change
   A_PosSpindle : BOOL ;    //Position spindle
   f30_5 : BOOL ;
   f30_6 : BOOL ;
   f30_7 : BOOL ;
   f31_0 : BOOL;
   f31_1 : BOOL;
   f31_2 : BOOL;
   f31_3 : BOOL;
   A_Resynchronize : BOOL;    // Resynchronize
   A_DisSync : BOOL;          // Disable synchronization
   A_Tracksync : BOOL;        // Track synchronism
   A_DelSyncRunCorr : BOOL;      // Deleting synchronous run correction
   f32_0 : BOOL ;
   f32_1 : BOOL ;
   A_extStopA : BOOL ;           //Deselection external Stop A
   A_extStopC : BOOL ;           //Deselection external Stop C
   A_extStopD : BOOL ;           //Deselection external Stop D
   A_extStopE : BOOL ;           //Deselection external Stop E
   f32_6 : BOOL ;
   f32_7 : BOOL ;
   f33_0 : BOOL ;
   f33_1 : BOOL ;
   f33_2 : BOOL ;
   f33_3 : BOOL ;
   A_SGcorr_0 : BOOL ;          //Selection SG-correction Bit 0
   A_SGcorr_1 : BOOL ;          //Selection SG-correction Bit 1
   A_SGcorr_2 : BOOL ;          //Selection SG-correction Bit 2
   A_SGcorr_3 : BOOL ;          //Selection SG-correction Bit 3
   A_SI_SetpLimBit0 : BOOL;     // Set point limitation Bit0
   A_SI_SetpLimBit1 : BOOL;     // Set point limitation Bit1
   f34_2 : BOOL;
   f34_3 : BOOL;
   f34_4 : BOOL;
   f34_5 : BOOL;
   f34_6 : BOOL;
   f34_7 : BOOL;
   f35  : BYTE;

   f36 : ARRAY  [36 .. 55 ] OF BYTE ;
   A_FeedDriveCAxEng : BOOL;  // Seperate feed drive as C axis engaged
   A_SpSpeedDisp : BOOL;      // Spindle speed display
   A_SpInsideClamp : BOOL;    // Spindle inside clamping
   f56_3 : BOOL;
   f56_4 : BOOL;
   f56_5 : BOOL;
   f56_6 : BOOL;
   f56_7 : BOOL;
   f57 : BYTE;
   f58 : WORD;    // FC18: internal
   E_SpNA : BOOL ;  //Spindle/no axis
   E_NCU_Link : BOOL ;  //NCU_link active axis
   E_EncodFreq1 : BOOL ;    //Encoder limit frequency 1 exceeded
   E_EncodFreq2 : BOOL ;    //Encoder limit frequency 2 exceeded
   E_RefSyn1 : BOOL ;   //Referenced/synchronized 1
   E_RefSyn2 : BOOL ;   //Referenced/synchronized 2
   E_ExactCoarse : BOOL ;   //Position reached with exact stop coarse
   E_ExactFine : BOOL ; //Position reached with exact stop fine
   E_TravRequ : BOOL ;  //Travel request
   E_AxialAlarm : BOOL ;   // Axial alarm
   E_AxisReady : BOOL ; //Axis ready
   E_Follow_upMode : BOOL ; //Follow-up mode active
   E_Stat : BOOL ;  //Axis/spindle stationary (n<nmin)
   E_PositContr : BOOL ;    //Position controller active
   E_SpeedContr : BOOL ;    //Speed controller active
   E_CurrentContr : BOOL ;  //Current controller active
   E_SWCam : BOOL ; //Software cams active
   E_HWOverlay : BOOL ; //Handwheel overlay active
   E_RevFD : BOOL ; //Revolutional feedrate active
   E_MeasAct : BOOL ;   //Measuring active
   E_ActTravFStop : BOOL ;  //Activate travel to fixed stop
   E_FixedStop : BOOL ; //Fixed stop reached
   E_ForceFixedStop : BOOL;      // Force fixed stop limited
   E_AxContainerRot : BOOL;      // Axis container rotation active
   E_AxReset : BOOL;          // Axis reset done
   E_PLCCtrlAx : BOOL;        // PLCcontrolled axis
   E_AxStop : BOOL;           // Axis stop active
   E_AxSpDisable : BOOL;      // Axis/spindle disable active
   E_StopDEPMCS : BOOL;       // stop DEPMCS active
   E_StopDEPBCS : BOOL;       // stop DEPBCS active
   E_StopCorr : BOOL;         // stop Corr active
   E_StopHIAxMove : BOOL;     // Stop HIAxMove active
   E_HW1 : BOOL ;   //Handwheel 1 active
   E_HW2 : BOOL ;   //Handwheel 2 active
   E_HW3 : BOOL ;   //Handwheel 3 active
   f64_3 : BOOL ;
   E_TReqMinus : BOOL ;   // Travel request minus
   E_TReqPlus : BOOL ;   // Travel request plus
   E_TCMinus : BOOL ;   //Traverse command minus
   E_TCPlus : BOOL ;    //Traverse command plus
   E_INC1 : BOOL ;  //INC1
   E_INC10 : BOOL ; //INC10
   E_INC100 : BOOL ;    //INC100
   E_INC1000 : BOOL ;   //INC1000
   E_INC10000 : BOOL ;  //INC10000
   E_INCVar : BOOL ;    //INC variable
   f65_6 : BOOL;
   f65_7 : BOOL;
   E_OEMAxis : BYTE ;   //OEM axis signals
   E_InvHWDirOfRot : BOOL;    // Handwheel direction of rotation invert actively
   f67_1 : BOOL;
   f67_2 : BOOL;
   f67_3 : BOOL;
   f67_4 : BOOL;
   f67_5 : BOOL;
   f67_6 : BOOL;
   f67_7 : BOOL;
   E_NCASpChanA : BOOL ;    //NC axis/spindle in channel A
   E_NCASpChanB : BOOL ;    //NC axis/spindle in channel B
   E_NCASpChanC : BOOL ;    //NC axis/spindle in channel C
   E_NCASpChanD : BOOL ;    //NC axis/spindle in channel D
   E_PLCType : BOOL ;   //New type requested by PLC
   E_ChPoss : BOOL ;    //Change axis possible
   E_NeutrASp : BOOL ;  //Neutral axis/spindle
   E_PLCASp : BOOL ;    //PLC axis/spindle
   E_ParS_A : BOOL ;    //Parameter block servo A
   E_ParS_B : BOOL ;    //Parameter block servo B
   E_ParS_C : BOOL ;    //Parameter block servo C
   E_NCUNumLink_3 : BOOL;
   E_NCUNumLink_4 : BOOL;
   E_NCUNumLink_5 : BOOL;
   E_NCUNumLink_6 : BOOL;
   E_NCUNumLink_7 : BOOL;
   E_ReposSh : BOOL ;      // Repos shift
   E_ReposShValid : BOOL;     // Repos shift valid
   E_ReposDelayQuit : BOOL;   // Repos delay quit
   f70_3 : BOOL;
   E_SI_Nck : BOOL;         // NCK-Safety Integrated active
   E_SI_Drv_SICSCC : BOOL;  // DRV-Safety Integrated with SIC/SCC active
   f70_6 : BOOL;
   f70_7 : BOOL;
   E_BrakeTest: BOOL;         // Brake test active
   f71_1 : BOOL;
   f71_2 : BOOL;
   f71_3 : BOOL;
   E_POS_RESTORED1 : BOOL;    // POS_RESTORED 1
   E_POS_RESTORED2 : BOOL;    // POS_RESTORED 2
   f71_6 : BOOL;
   E_PLCAxDedic : BOOL;       // PLC Axis dedicated
   E_MMC_REPOSDelay : BOOL ;    //MMC REPOS DELAY
   f72_1 : BOOL ;
   f72_2 : BOOL ;
   f72_3 : BOOL ;
   f72_4 : BOOL ;
   f72_5 : BOOL ;
   f72_6 : BOOL ;
   f72_7 : BOOL ;
   f73 : BYTE ;
   f74_0 : BOOL;
   f74_1 : BOOL;
   f74_2 : BOOL;
   f74_3 : BOOL;
   E_ModLimEnAct : BOOL;      // Modulo limit enabled active
   f74_5 : BOOL;
   f74_6 : BOOL;
   f74_7 : BOOL;
   E_JogFixPPos0Act     : BOOL ;    // JogFixPointPos 0 active
   E_JogFixPPos1Act     : BOOL ;    // JogFixPointPos 1 active
   E_JogFixPPos2Act     : BOOL ;    // JogFixPointPos 2 active
   E_JogFixPPos0        : BOOL ;    // JogFixPointPos 0 reached
   E_JogFixPPos1        : BOOL ;    // JogFixPointPos 1 reached
   E_JogFixPPos2        : BOOL ;    // JogFixPointPos 2 reached
   E_JogToPos           : BOOL ;    // Jog to position active
   E_JogPos             : BOOL ;    // Jog position reached
   E_ScratchPulse : BOOL ;  //Scratch pulse
   f76_1 : BOOL ;
   f76_2 : BOOL ;
   f76_3 : BOOL ;
   E_PathAxis : BOOL ;        // Path axis
   E_PosAxis : BOOL ;   //Positioning axis
   E_IndexAxisPos : BOOL ;  //Indexing axis in position
   E_CurvePos : BOOL ;  //Curve axis in position
   E_CollCheckRedSpeed : BOOL; //reduced speed of Collisions Check
   f77_1 : BOOL ;
   f77_2 : BOOL ;
   f77_3 : BOOL ;
   f77_4 : BOOL ;
   f77_5 : BOOL ;
   f77_6 : BOOL ;
   f77_7 : BOOL ;
   E_FPosAxis : REAL ;  //F function (REAL format) for positioning axes
   E_SetpGearA : BOOL ; //Setpoint gear stage A
   E_SetpGearB : BOOL ; //Setpoint gear stage B
   E_SetpGearC : BOOL ; //Setpoint gear stage C
   E_GearChange : BOOL ;    //Gear changeover
   f82_4 : BOOL ;
   f82_5 : BOOL ;
   f82_6 : BOOL ;
   f82_7 : BOOL ;
   E_SpeedLimit : BOOL ;    //Speed limit exceeded
   E_SetSpeedLimit : BOOL ; //Setpoint speed limited
   E_SetSpeedIncreased : BOOL ; //Setpoint speed increased
   E_GeoMonit : BOOL ;  //Geometry monitoring
   E_SupportAreaViol : BOOL ;   //Support area limits violated
   E_SetRange : BOOL ;  //Spindle in setpoint range
   E_SpeedMonit : BOOL ;    //Speed monitoring
   E_ActRotRight : BOOL ;   //Actual rotation direction right
   E_ConstCuttSpeed : BOOL ;    //Const. cutting speed active
   E_SUG : BOOL ;   //SUG active (grinding wheel surface speed)
   E_CLG : BOOL ;   //CLG active
   E_Tapping : BOOL ;   //Tapping without compensating chuck
   E_SyncMode : BOOL ;  //Synchronous mode spindle active
   E_PosMode : BOOL ;   //Positioning mode spindle active
   E_OscillMode : BOOL ;    //Oscillation mode spindle active
   E_ContrMode : BOOL ; //Control mode spindle active
   E_ToolDynLimit : BOOL;     // Tool with limit of dynamics
   f85_1 : BOOL;
   f85_2 : BOOL;
   f85_3 : BOOL;
   f85_4 : BOOL;
   E_SpInPosition : BOOL;     // Spindle in position
   f85_6 : BOOL;
   f85_7 : BOOL;
   E_MFunct : INT ; //M function (INT) for spindle
   E_SFunct : REAL ;    //S function (REAL) for spindle
   f92_0    : BOOL;
   E_RUEncDisabl : BOOL ;           //Run-up encoder disable active
   f92_2    : BOOL;
   E_SpeedSetpSmooth : BOOL ;       //Speed setpoint smoothing active
   E_RLIact : BOOL ;                // RLI active
   E_HoldBrakeOpened : BOOL ;       // Holding brake opened
   f92_6 : BOOL ;
   E_DriveRunEn : BOOL ;            // Drive run enabled
   E_ParA : BOOL ;  //Active parameter set A
   E_ParB : BOOL ;  //Active parameter set B
   E_ParC : BOOL ;  //Active parameter set C
   E_MotA : BOOL ;  //Active motor A
   E_MotB : BOOL ;  //Active motor B
   E_MotOK : BOOL ; //Drive ready
   E_IntegratDisable : BOOL ;   //n controller integrator disabled
   E_PulseEnable : BOOL ;   //Pulses enabled
   E_MTempWarn : BOOL ; //Temperature prewarning motor
   E_HTempWarn : BOOL ; //Temperature prewarning heat sink
   E_RUComplete : BOOL ;    //Ramp-up complete
   E_MdMdx : BOOL ; //Md<Mdx
   E_NactNmin : BOOL ;  //nact<nmin
   E_NactNx : BOOL ;    //nact<nx
   E_NactNset : BOOL ;  //nact=nset
   E_Message : BOOL ;   //Variable message function
   E_UDClessAlThreshold : BOOL ;    //UDC-link < alarm threshold
   f95_1 : BOOL;
   f95_2 : BOOL;
   f95_3 : BOOL;
   f95_4 : BOOL;
   f95_5 : BOOL;
   f95_6 : BOOL;
   E_I2TLimit : BOOL;   // Power Section I2T limit
   E_SpindleMonit : BOOL ;  //Error spindle monitoring
   E_AxisCtrl : BOOL ;              // Axis control active
   E_MSFine : BOOL ;                // Master/Slave fine
   E_MSCoarse : BOOL ;              // Master/Slave coarse
   E_MSCompContr : BOOL ;           // Master/Slave Compensation controller activ
   E_BitValCtrlOutChang0 : BOOL ;   // Bit value for CTRLOUT_changed 0:  Change setpoint output assignment
   E_BitValCtrlOutChang1 : BOOL ;   // Bit value for CTRLOUT_changed 1:  Change setpoint output assignment
   E_MS : BOOL ;    //Master/ slave active
   f97 : BYTE ;
   E_SyncronFine : BOOL ;   //Synchronism fine
   E_SyncronCoarse : BOOL ; //Synchronism coarse
   E_ActValCoupling : BOOL ;    //Actual value coupling
   f98_3 : BOOL ;
   E_OverlayMotion : BOOL ; //Overlaid motion
   E_SWL : BOOL ;   //Speed warning limit reached
   E_AWL : BOOL ;   //Acceleration warning limit reached
   E_EmRetr : BOOL ;    //Emergency retraction active
   E_MasterSp : BOOL ;  //Master spindle
   E_SlaveSp : BOOL ;   //Slave spindle
   E_SyncRunCorrDOut : BOOL ;    // Synchronous run correction driven out
   E_AxisAccel : BOOL ; //Axis accelerated
   E_Sync : BOOL ;  //Synchronization active
   E_MSR : BOOL ;   //Max speed reached
   E_MAR : BOOL ;   //Max acceleration reached
   f99_7 : BOOL ;
   f100_0 : BOOL ;
   f100_1 : BOOL ;
   E_OscillAxExtRev : BOOL ;  // OscillAxExt Reversal active
   E_StopOscill : BOOL ;    //Oscillation cannot start
   E_ErrorOscill : BOOL ;   //Error during oscillation
   E_SparkOut : BOOL ;  //Spark-out active
   E_OscillMotion : BOOL ;  //Oscillation motion active
   E_Oscill : BOOL ;    //Oscillation active
   f101_0 : BOOL ;
   f101_1 : BOOL ;
   E_GantCOLimit : BOOL ;   //Gantry cut-off limit exceeded
   E_GantWarn : BOOL ;  //Gantry warning limit exceeded
   E_SynRunStart : BOOL ;   //Synchronization run ready to start
   E_GantGroupSyn : BOOL ;  //Gantry grouping is synchronous
   E_GantLeadAxis : BOOL ;  //Gantry leading axis
   E_GantAxis : BOOL ;  //Gantry axis
   E_DynBComp : BOOL;   // dynamic backlash compensation activ
   f102_1 : BOOL ;
   f102_2 : BOOL ;
   E_ClampTolerance : BOOL;     //clamp tolerance exceeded
   f102_4 : BOOL ;
   E_PosMeas1 : BOOL ;  //Position measuring system 1 active
   E_PosMeas2 : BOOL ;  //Position measuring system 2 active
   f102_7 : BOOL ;
   E_SyncRunCorrIncl : BOOL;  // Synchronous run correction is included
   f103_1            : BOOL;
   f103_2            : BOOL;
   f103_3            : BOOL;
   E_Syncron2Fine : BOOL ;   //Synchronism fine
   E_Syncron2Coarse : BOOL ; //Synchronism coarse
   f103_6            : BOOL;
   f103_7            : BOOL;
   E_AIAxis : ARRAY  [1 .. 31 ] OF BOOL ;   //Active infeed axis[1..31]
   E_SG_SBH : BOOL ;    //Active SG/SBH
   E_ErrLifeS_CRC : BOOL ;    // Error lifesign or CRC-error
   E_ImpdelNCK : BOOL ; //Delete pulses NCK
   r108_3 : BOOL ;
   r108_4 : BOOL ;
   r108_5 : BOOL ;
   r108_6 : BOOL ;
   E_SRef : BOOL ;  //Axis safely referenced
   E_SN1Plus : BOOL ;   //Actual position > cam position SN1+
   E_SN1Minus : BOOL ;  //Actual position > cam position SN1-
   E_SN2Plus : BOOL ;   //Actual position > cam position SN2+
   E_SN2Minus : BOOL ;  //Actual position > cam position SN2-
   E_SN3Plus : BOOL ;   //Actual position > cam position SN3+
   E_SN3Minus : BOOL ;  //Actual position > cam position SN3-
   E_SN4Plus : BOOL ;   //Actual position > cam position SN4+
   E_SN4Minus : BOOL ;  //Actual position > cam position SN4-
   f110_0 : BOOL ;
   E_SBH : BOOL ;   //Active SBH
   f110_2 : BOOL ;
   E_SG_0 : BOOL ;  //Active SG 0
   E_SG_1 : BOOL ;  //Active SG 1
   E_n_nx : BOOL ;  //n < nx
   f110_6 : BOOL ;
   f110_7 : BOOL ;
   f111_0 : BOOL ;
   f111_1 : BOOL ;
   f111_2 : BOOL ;
   f111_3 : BOOL ;
   E_StopAB : BOOL ;    //Stop A/B active
   E_StopC : BOOL ; //Stop C active
   E_StopD : BOOL ; //Stop D active
   E_StopE : BOOL ; //Stop E active

   E_CamRangeTr1 : BYTE;      //Cam Range for Cam Track 1
   E_CamRangeTr2 : BYTE;      //Cam Range for Cam Track 2
   E_CamRangeTr3 : BYTE;      //Cam Range for Cam Track 3
   E_CamRangeTr4 : BYTE;      //Cam Range for Cam Track 4
   f116 : BYTE;
   E_CamTrack1 : BOOL;        //Cam Track 1
   E_CamTrack2 : BOOL;        //Cam Track 2
   E_CamTrack3 : BOOL;        //Cam Track 3
   E_CamTrack4 : BOOL;        //Cam Track 4
   f117_4 : BOOL;
   f117_5 : BOOL;
   f117_6 : BOOL;
   f117_7 : BOOL;
   E_CamRangeBitTr1 : ARRAY  [0 .. 14 ] OF //Cam Range Bits for Cam Track 1
    BOOL ;
   E_CamRangeBitTr2 : ARRAY  [0 .. 14 ] OF //Cam Range Bits for Cam Track 2
    BOOL ;
   E_CamRangeBitTr3 : ARRAY  [0 .. 14 ] OF //Cam Range Bits for Cam Track 3
    BOOL ;
   E_CamRangeBitTr4 : ARRAY  [0 .. 14 ] OF //Cam Range Bits for Cam Track 4
    BOOL ;
   f126           : WORD;        // internal
   E_MMC_ProgtestSuppress  : BOOL;  // HMI->PLC: Program test to supress
   E_MMC_ProgtestActivate  : BOOL;  // HMI->PLC: Program test activate
   f128_2            : BOOL;
   f128_3            : BOOL;
   f128_4            : BOOL;
   f128_5            : BOOL;
   f128_6            : BOOL;
   f128_7            : BOOL;
   f129              : BYTE;
   f130              : WORD;
   E_SensorAv        : BOOL;     // Sensors available
   E_S1aMeasARod     : BOOL;     // Sensor S1: analogous measurement position of actuating rod
   f132_2            : BOOL;
   f132_3            : BOOL;
   E_S4dPistonStopP  : BOOL;     // Sensor S4: digital value piston stop position
   E_S5dAngleShaft   : BOOL;     // Sensor S5: digital value angle situation shaft
   E_S6Temp          : BOOL;     // Sensor S6:temperature
   f132_7            : BOOL;
   f133              : BYTE;
   E_ClampingState   : INT;      // state of the clamping system
   E_AnalogSensor    : INT;      // analog sensor on the motor
   f138_0            : BOOL;
   f138_1            : BOOL;
   f138_2            : BOOL;
   f138_3            : BOOL;
   E_S4PistonStopP   : BOOL;     // Sensor S4: piston stop position
   E_S5AngleShaft    : BOOL;     // Sensor S5: angle situation shaft
   f138_6            : BOOL;
   f138_7            : BOOL;
   f139              : BYTE;

   SCC : STRUCT  //PLC to Drive (SCC)
     CW1 : STRUCT
        TeststopStart   : BOOL; // Teststops for extended functionen
        res140_1        : BOOL;
        res140_2        : BOOL;
        res140_3        : BOOL;
        res140_4        : BOOL;
        res140_5        : BOOL;
        res140_6        : BOOL;
        res140_7        : BOOL;
        res141          : BYTE;
     END_STRUCT ;
     CW3 : STRUCT
        res142          : BYTE;
        SelectionSBT    : BOOL; // Selection: safe brake test
        BT_Start        : BOOL; // Start: brake test
        Brake_1_2       : BOOL; // brake test with brake 1 or 2
        DirOfROT        : BOOL; // Direction of rotation
        Testseq_1_2     : BOOL; // Testsequence 1 or 2
        BrakeClosed     : BOOL; // Feedback external brake
        res143_6        : BOOL;
        res143_7        : BOOL;
     END_STRUCT ;
   END_STRUCT ;
   res144_163 : ARRAY  [144 .. 163 ] OF BYTE;

   SIC : STRUCT  //Drive to PLC (SIC)
     SW1 : STRUCT
        res164_0        : BOOL;
        SLS_LimBit0_Sel : BOOL; // Safely-Limited Speed: limit Bit0 selected
        SLS_LimBit1_Sel : BOOL; // Safely-Limited Speed: limit Bit1 selected
        res164_3        : BOOL;
        res164_4        : BOOL;
        res164_5        : BOOL;
        ESR_Req         : BOOL; // Extended Stop and Retract requested
        SF_Message_Act  : BOOL; // Safety error active
        STO_Act         : BOOL; // Safe torque off: active
        SS1_Act         : BOOL; // Safe Stop1: active
        SS2_Act         : BOOL; // Safe Stop2: active
        SOS_Act         : BOOL; // Safe Operating Stop: active
        SLS_Act         : BOOL; // Safely-Limited Speed: active
        SOS_Sel         : BOOL; // Safe Operating Stop: selected
        SLS_Sel         : BOOL; // Safely-Limited Speed: selected
        InternalEvent   : BOOL; // Safety error with Stop A active
     END_STRUCT ;
     SW2 : STRUCT
        SDI_P_Sel       : BOOL; // Safe direction positiv: selected
        SDI_N_Sel       : BOOL; // Safe direction negativ: selected
        res166_2        : BOOL;
        res166_3        : BOOL;
        TestStopAct     : BOOL; // Teststop active
        TestStopReq     : BOOL; // Teststop requested
        res166_6        : BOOL;
        res166_7        : BOOL;
        res167_0        : BOOL;
        res167_1        : BOOL;
        res167_2        : BOOL;
        res167_3        : BOOL;
        SLP_LimBit0_Sel : BOOL; // Safely-Limited Position: limit Bit0 selected
        res167_5        : BOOL;
        res167_6        : BOOL;
        SLP_Sel         : BOOL; // Safely-Limited Position: selected
     END_STRUCT ;
     V_Limit_B          : DINT; // Setpoint speed limit effective
     SW3 : STRUCT
        res172_0        : BOOL;
        res172_1        : BOOL;
        res172_2        : BOOL;
        res172_3        : BOOL;
        res172_4        : BOOL;
        res172_5        : BOOL;
        AcceptSLPAct    : BOOL; // Acceptance test Safely-Limited Position active
        AcceptTestSel   : BOOL; // Acceptance test selected
        SBT_Sel         : BOOL; // Safety break test: selected
        SetpSettingDrive : BOOL; // Setpoint input is in the drive during the SBT
        Brake_1_2       : BOOL; // Test with brake 1 or 2
        BT_Act          : BOOL; // Brake test: active
        BT_OK           : BOOL; // Brake test: ok
        BT_Finished     : BOOL; // Brake test: finished
        BrakeReq        : BOOL; // External brake close requested
        SignLoadTorque  : BOOL; // Sign of load torque is negative
     END_STRUCT ;
  END_STRUCT;
  res174_187 : ARRAY  [174 .. 187 ] OF BYTE;

  END_STRUCT ;



END_TYPE


//***** UDT 77 *****
TYPE UDT 77
//**************************************************************************
//if MCPs via Standard-SDB210 (only 840Di)

     STRUCT
   MCP1In: ARRAY  [0 .. 7 ] OF BYTE;
   MCP1Out: ARRAY  [0 .. 7 ] OF BYTE;
   MCP1StatSend: DWORD;
   MCP1StatRec: DWORD;
   MCP2In: ARRAY  [0 .. 7 ] OF BYTE;
   MCP2Out: ARRAY  [0 .. 7 ] OF BYTE;
   MCP2StatSend: DWORD;
   MCP2StatRec: DWORD;

   BHGIn: ARRAY  [0 .. 5 ] OF BYTE;
   Filler: ARRAY  [0 .. 5 ] OF BYTE;
   BHGOut: ARRAY  [0 .. 19 ] OF BYTE;
   BHGStatSend: DWORD;
   BHGStatRec: DWORD;
   END_STRUCT ;


END_TYPE



//***** UDT 1002 *****
TYPE UDT 1002

    STRUCT
//Offset 0
   Chan : ARRAY [1 .. 10] OF STRUCT     //From Channel 1 to Channel 10
    FDD : ARRAY  [0 .. 15 ] OF //Feed disable
    BOOL ;
    RID : ARRAY  [0 .. 15 ] OF //Read-in disable
    BOOL ;
    NCSD : ARRAY  [0 .. 15 ] OF //NC start disable
    BOOL ;
    FdStop_1 : ARRAY  [0 .. 15 ] OF //Feed stop GEOaxis 1
    BOOL ;
    FdStop_2 : ARRAY  [0 .. 15 ] OF //Feed stop GEOaxis 2
    BOOL ;
    FdStop_3 : ARRAY  [0 .. 15 ] OF //Feed stop GEOaxis 3
    BOOL ;
   END_STRUCT ;
//without Alarmno for Chan (120 Byte)
//Offset 120
    Axis : ARRAY [1 .. 31] OF STRUCT  //From Axis 1 to Axis 31
    FdStop : ARRAY  [0 .. 15 ] OF //Feed stop axis/spindle 1
    BOOL ;
   END_STRUCT ;
//without Alarmno for Axis (62 Byte)
//Offset 182
   ZInfo0 : ARRAY [0 .. 63] OF WORD; //Additional Value for UserAlarms 700000 to 700063
//Offset 310

   ChanA : ARRAY [1 .. 10] OF STRUCT    //From Channel 1 to Channel 10
    FDD_5C00xx : ARRAY  [0 .. 15 ] OF //Feed disable A.no.51000-510015
    BOOL ;
    FDD_RID_5C01xx : ARRAY  [0 .. 31 ] OF //Feed and read-in disable A.no.510100-510131
    BOOL ;
    RID_5C02xx : ARRAY  [0 .. 31 ] OF //Read-in disable A.no.510200-510231
    BOOL ;
    NCSD_5C03xx : ARRAY  [0 .. 15 ] OF //NC start disable A.no.510300-510315
    BOOL ;
    FdStop_1_5C11xx : ARRAY  [0 .. 15 ] OF //Feed stop GEOaxis 1 A.no.511100-511115
    BOOL ;
    FdStop_2_5C12xx : ARRAY  [0 .. 15 ] OF //Feed stop GEOaxis 2 A.no.511200-511215
    BOOL ;
    FdStop_3_5C13xx : ARRAY  [0 .. 15 ] OF //Feed stop GEOaxis 3 A.no.511300-511315
    BOOL ;
   END_STRUCT ;
//Alarmno for Chan are 5Cxxxx; C is the ChannelNo, except Channel 10. Channel 10 has a value C = 0
//(180Byte)
//Offset 490
    AxisA : ARRAY [1 .. 32] OF STRUCT  //From Axis 1 to Axis 31
    AAFdStop60AAxx : ARRAY  [0 .. 15 ] OF //Feed stop axis/spindle
    BOOL ;
   END_STRUCT ;
//Alarmno for Axis are 60AAxx; A is the Axisno.
//Offset 554
   UserA : ARRAY [0 .. 63] OF STRUCT
   A70UUxx : ARRAY  [0 .. 63 ] OF //Alarm 700000-700063 (user area 0)
   BOOL ;
   END_STRUCT ;
//Alarmno for UserAlarms are 7yUUxx; U is the Userarea, y = Db1004.UserDek2No[U]
  END_STRUCT ;


END_TYPE

//SIN_SL


